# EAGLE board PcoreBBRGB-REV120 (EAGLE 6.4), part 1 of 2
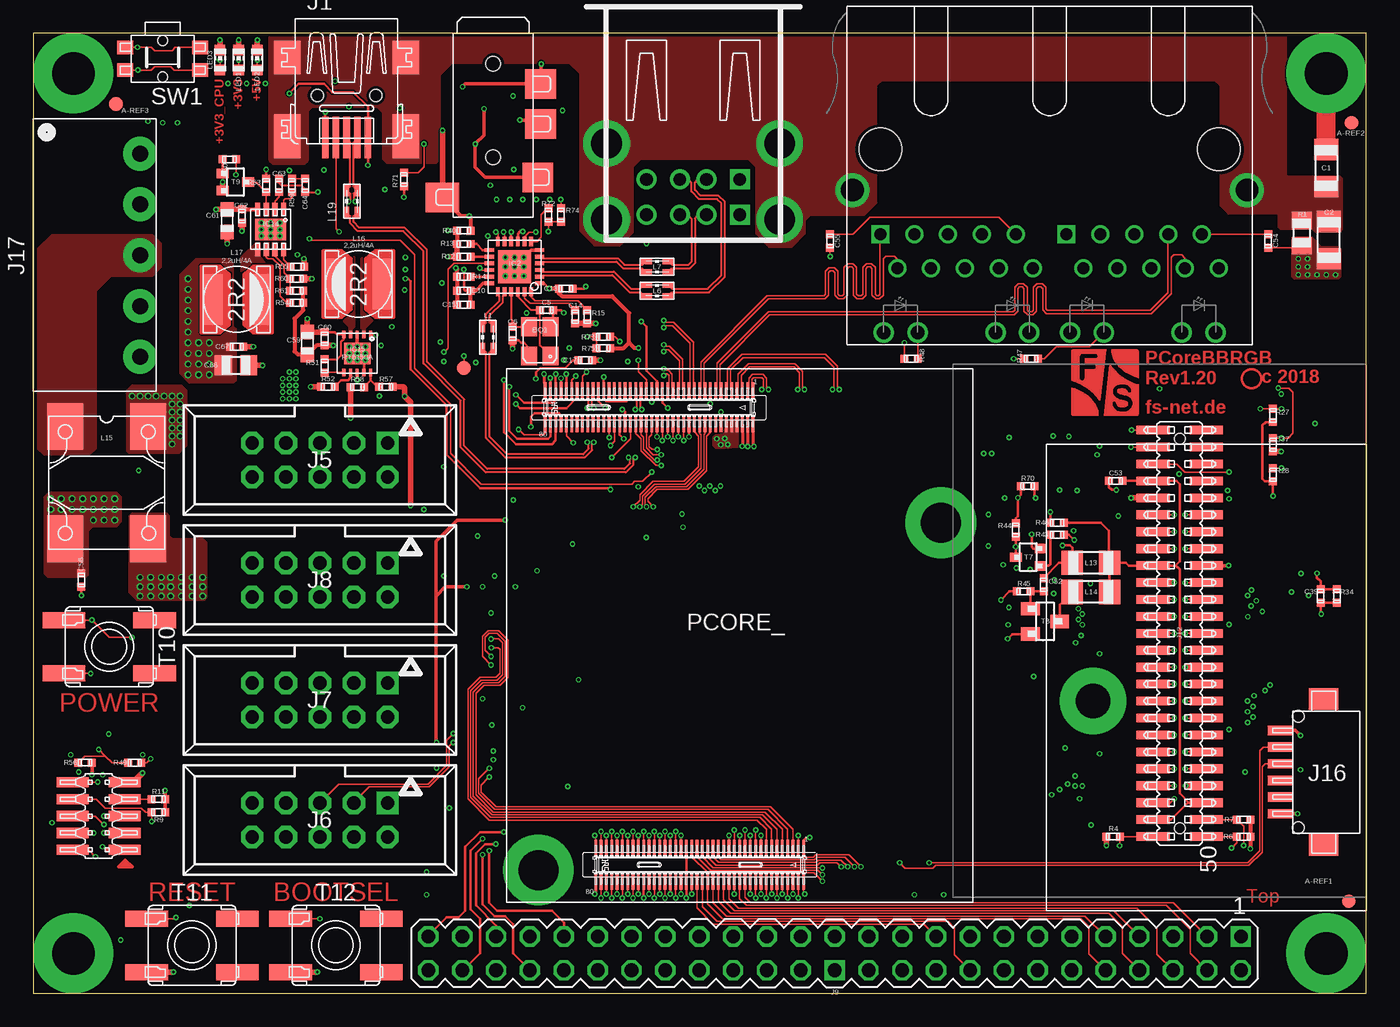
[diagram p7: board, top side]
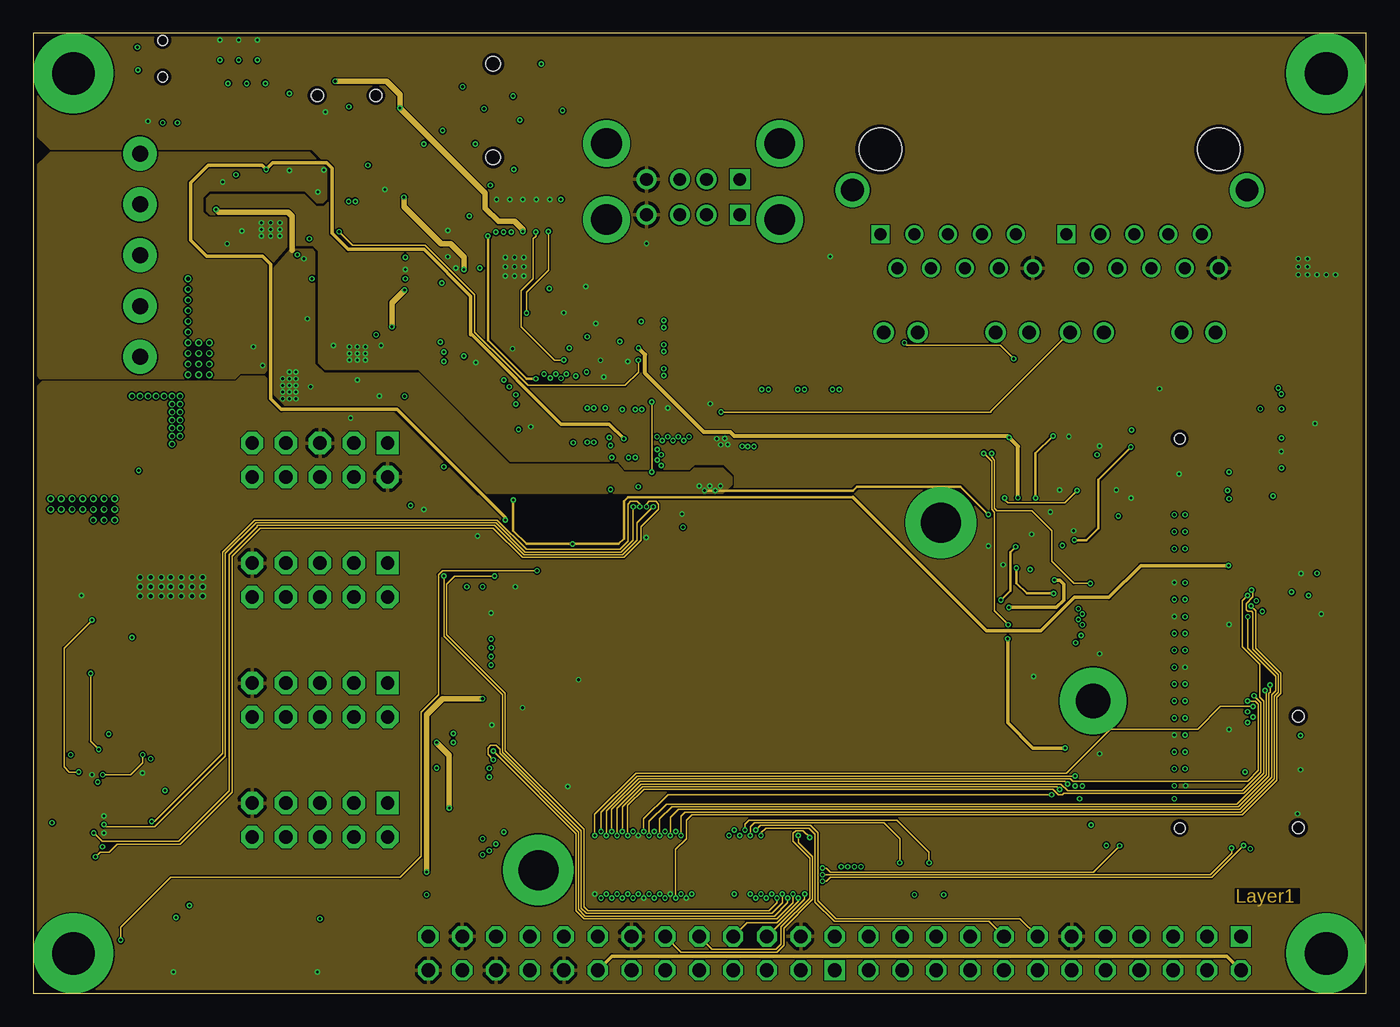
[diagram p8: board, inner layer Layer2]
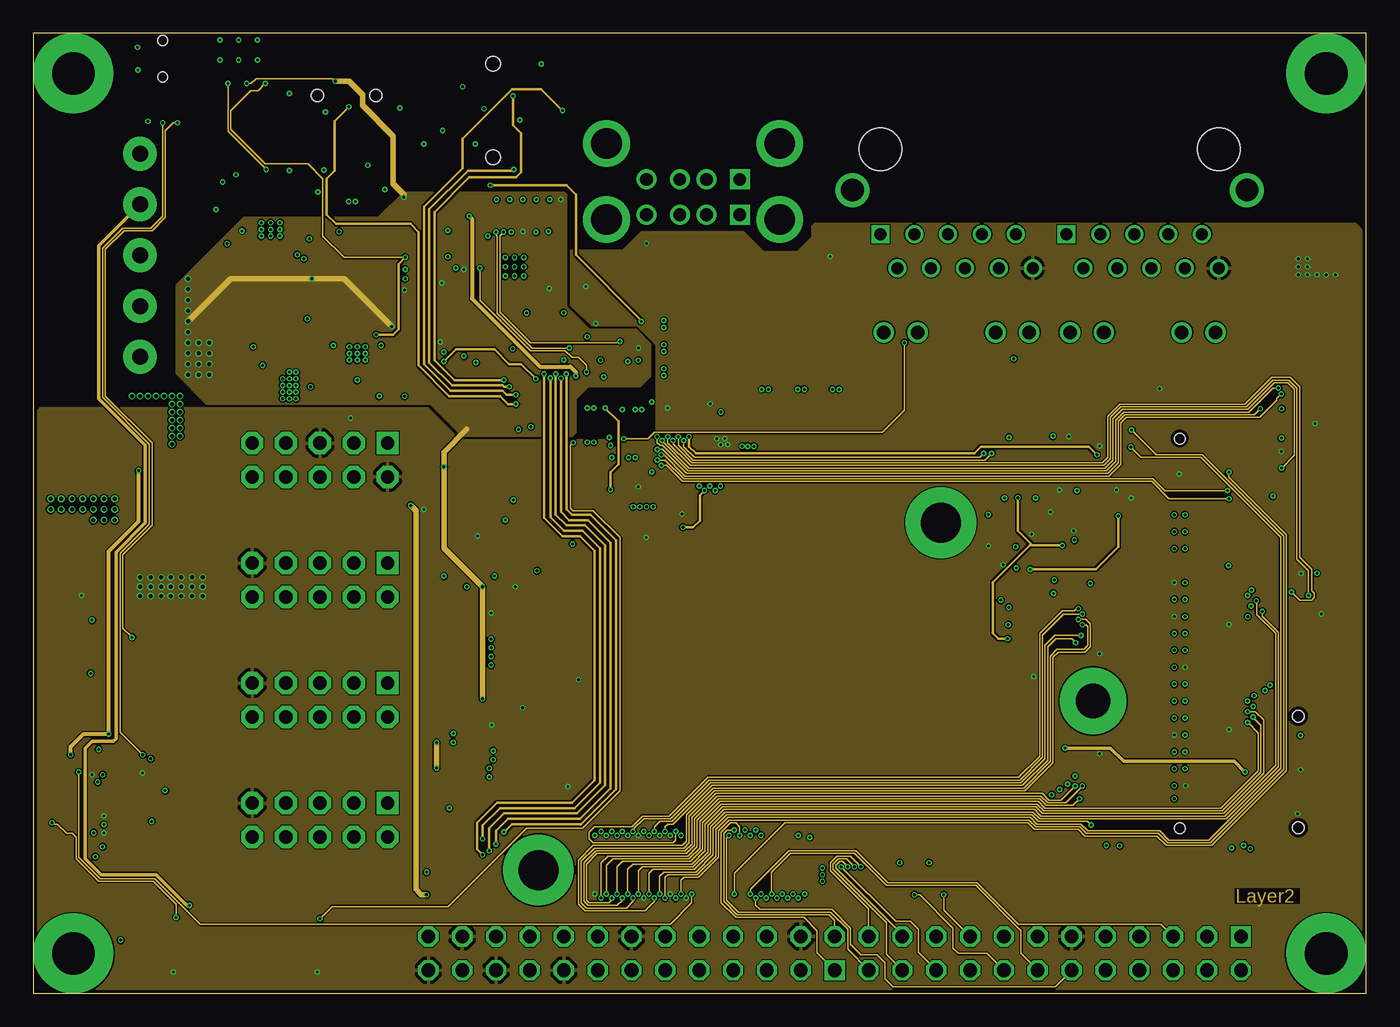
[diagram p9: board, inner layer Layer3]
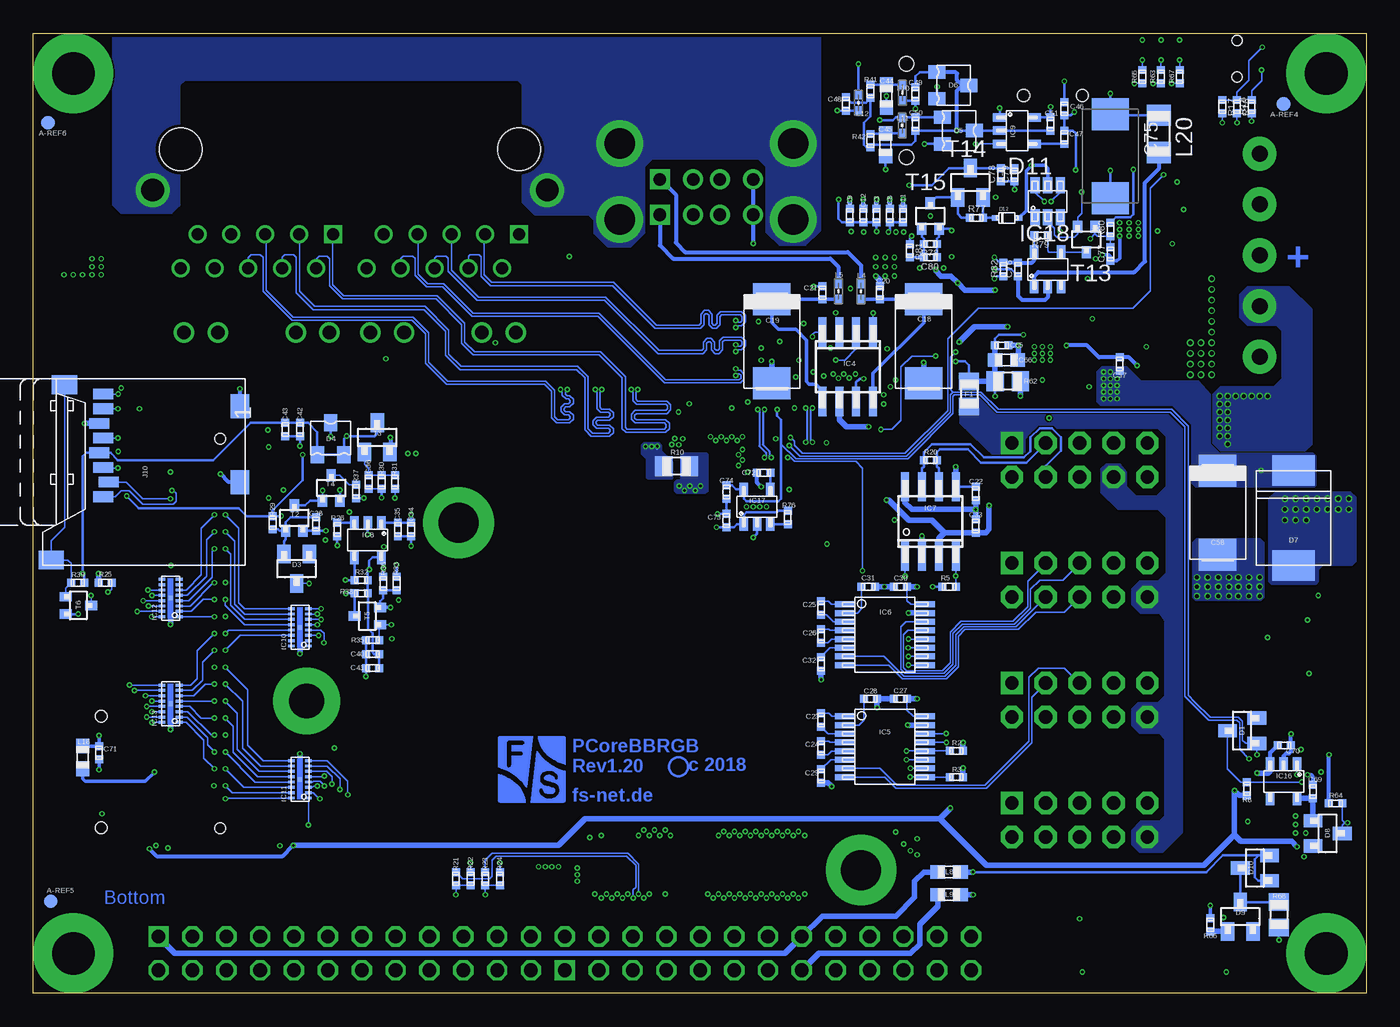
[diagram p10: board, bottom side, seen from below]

Size 100 x 72 mm. Coordinates in mm from the lower left corner, seen from the top.
Outline: 0,0 100,0 100,72 0,72 0,0
Copper layers (1*2*15*16): Top 0.035mm / dielectric 0.14mm / Layer2 0.035mm / dielectric 1.2mm / Layer3 0.035mm / dielectric 0.14mm / Bottom 0.035mm
Design rules "default *": minimum track width 0.1mm, minimum drill 0.2mm, track to track 0.1mm, track to pad 0.1mm, pad to pad 0.1mm, via to via 0.1mm, smd to smd 0.1mm, copper to edge 10mil, drill to drill 8mil, minimum pad ring 0.1mm, minimum via ring 0.1mm, stop-mask expansion 0mil, vias tented up to drill 0.6mm, thermal gap 10mil
Net classes: 0 default: width 0.1 mm, drill 0.2 mm, clearance 0.1 mm; 1 USB: width 0.161 mm, drill 0.2 mm, clearance 0.5 mm to class 0, clearance 0.1 mm; 2 ETHERNET: width 0.127 mm, drill 0.2 mm, clearance 0.5 mm to class 0, clearance 0.5 mm to class 1, clearance 0.1 mm; 3 +3V3: width 0.1 mm, drill 0.2 mm, clearance 0.1 mm to class 0, clearance 0.5 mm to class 1, clearance 0.5 mm to class 2, clearance 0.1 mm

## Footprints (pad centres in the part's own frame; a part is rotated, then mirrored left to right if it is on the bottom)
A-REF = smd 1 x 1: P$1 0,0
FA-238 = smd 1.4 x 1.2: 1 -1.1,-0.8; 2 1.1,-0.8; 3 1.1,0.8; 4 -1.1,0.8
1206 = smd 1.6 x 1.803: 1 -1.4,0; 2 1.4,0
0402@2 = smd 0.6 x 0.6: 1 -0.5,0; 2 0.5,0
SMC_D@1 = smd 2.4 x 2.8: + -3.15,0; - 3.15,0
0603 = smd 1.1 x 1: 1 -0.85,0; 2 0.85,0
0805 = smd 1.3 x 1.5: 1 -0.95,0; 2 0.95,0
SMC_D = smd 2.4 x 2.8: + -3.15,0; - 3.15,0
SOT23 = smd 1 x 1.4: 1 -0.95,-1.1; 2 0.95,-1.1; 3 0,1.1
SOT-23 = smd 1 x 1.27: 1 -1,-1.2; 2 1,-1.2; 3 0,1.2
D-DO214AB(SMC) = smd 2.286 x 3.175: 1 -3.556,0; 2 3.556,0
SOT26 = smd 0.7 x 1.2: 1 -0.95,-1.2; 2 0,-1.2; 3 0.95,-1.2; 4 0.95,1.2; 5 0,1.2; 6 -0.95,1.2
SOD-523 = smd 0.48 x 0.4: 1 -0.9,0; 2 0.9,0
HOLE-3.2X6 = drill 3.2 pad 6: P$1 0,0
SQFN-24 = smd 0.28 x 0.69: 1 -1.25,-1.883; 2 -0.75,-1.883; 3 -0.25,-1.883; 4 0.25,-1.883; 5 0.75,-1.883; 6 1.25,-1.883; 13 1.25,1.883; 14 0.75,1.883; 15 0.25,1.883; 16 -0.25,1.883; 17 -0.75,1.883; 18 -1.25,1.883 | smd 0.69 x 0.28: 7 1.883,-1.25; 8 1.883,-0.75; 9 1.883,-0.25; 10 1.883,0.25; 11 1.883,0.75; 12 1.883,1.25; 19 -1.883,1.25; 20 -1.883,0.75; 21 -1.883,0.25; 22 -1.883,-0.25; 23 -1.883,-0.75; 24 -1.883,-1.25 | smd 2.5 x 2.5: 25 0,0
SO-8$1 = smd 0.6 x 2.2: 1 -1.905,-2.6; 2 -0.635,-2.6; 3 0.635,-2.6; 4 1.905,-2.6; 5 1.905,2.6; 6 0.635,2.6; 7 -0.635,2.6; 8 -1.905,2.6
TSSOP-16 = smd 0.45 x 1.5: 1 -2.275,-3; 2 -1.625,-3; 3 -0.975,-3; 4 -0.325,-3; 5 0.325,-3; 6 0.975,-3; 7 1.625,-3; 8 2.275,-3; 9 2.275,3; 10 1.625,3; 11 0.975,3; 12 0.325,3; 13 -0.325,3; 14 -0.975,3; 15 -1.625,3; 16 -2.275,3
SO-8 = smd 0.6 x 2.2: 1 -1.9,-2.6; 2 -0.635,-2.6; 3 0.635,-2.6; 4 1.9,-2.6; 5 1.9,2.6; 6 0.635,2.6; 7 -0.635,2.6; 8 -1.9,2.6
SOT23-5 = smd 0.635 x 1: 1 -1,-1.3; 2 0,-1.3; 3 1,-1.3; 4 1,1.3; 5 -1,1.3
SOT1168-1 = smd 0.22 x 0.5: 1 -1.4,-0.64; 2 -1,-0.64; 3 -0.6,-0.64; 4 -0.2,-0.64; 5 0.2,-0.64; 6 0.6,-0.64; 7 1,-0.64; 8 1.4,-0.64; 9 1.4,0.64; 10 1,0.64; 11 0.6,0.64; 12 0.2,0.64; 13 -0.2,0.64; 14 -0.6,0.64; 15 -1,0.64; 16 -1.4,0.64 | smd 0.35 x 0.3: 17 0,0
WDFN-8L = smd 0.4 x 1: 1 -0.975,-1.5; 2 -0.325,-1.5; 3 0.325,-1.5; 4 0.975,-1.5; 5 0.975,1.5; 6 0.325,1.5; 7 -0.325,1.5; 8 -0.975,1.5 | smd 2.35 x 1.6: 9 0,0
WDFN-10L3X3 = smd 0.23 x 0.55: 1 -1,-1.425; 2 -0.5,-1.425; 3 0,-1.425; 4 0.5,-1.425; 5 1,-1.425; 6 1,1.425; 7 0.5,1.425; 8 0,1.425; 9 -0.5,1.425; 10 -1,1.425 | smd 2 x 1.6: 11 0,0
SOT23-5@1 = smd 0.635 x 1: 1 -1,-1.3; 2 0,-1.3; 3 1,-1.3; 4 1,1.3; 5 -1,1.3
32005-201 = smd 0.5 x 3.1: 1 1.6,-8.918; 2 0.8,-8.918; 3 0,-8.918; 4 -0.8,-8.918; 5 -1.6,-8.918 | smd 2 x 2.5: M1 -4.45,-2.918; M2 4.45,-2.918 | smd 2 x 3.3: M3 4.45,-8.818; M4 -4.45,-8.818 | hole 0.9: -2.2,-5.768; 2.2,-5.768
10-POL.SMD-127 = smd 0.76 x 2.4: 1 -2.54,-1.95; 2 -2.54,1.95; 3 -1.27,-1.95; 4 -1.27,1.95; 5 0,-1.95; 6 0,1.95; 7 1.27,-1.95; 8 1.27,1.95; 9 2.54,-1.95; 10 2.54,1.95
LUMBERG-2410-03 = drill 0.95 pad 1.5 square: 1 12.96,3.5; 5 15.61,3.5 | drill 0.95 pad 1.5: 2 12.96,1; 3 12.96,-1; 4 12.96,-3.5; 6 15.61,1; 7 15.61,-1; 8 15.61,-3.5 | drill 2.3 pad 3.5: 9 10.26,6.5; 10 10.26,-6.5; 11 15.96,6.5; 12 15.96,-6.5
CON-10POL.-STIFTWANNE = drill 1 pad 1.676 square: 1 -5.08,-1.27 | drill 1 pad 1.676 octagon: 2 -5.08,1.27; 3 -2.54,-1.27; 4 -2.54,1.27; 5 0,-1.27; 6 0,1.27; 7 2.54,-1.27; 8 2.54,1.27; 9 5.08,-1.27; 10 5.08,1.27
50-POL. = drill 1.016 square: 1 -30.48,-1.27; 26 0,1.27 | drill 1.016 octagon: 2 -30.48,1.27; 3 -27.94,-1.27; 4 -27.94,1.27; 5 -25.4,-1.27; 6 -25.4,1.27; 7 -22.86,-1.27; 8 -22.86,1.27; 9 -20.32,-1.27; 10 -20.32,1.27; 11 -17.78,-1.27; 12 -17.78,1.27; 13 -15.24,-1.27; 14 -15.24,1.27; 15 -12.7,-1.27; 16 -12.7,1.27; 17 -10.16,-1.27; 18 -10.16,1.27; 19 -7.62,-1.27; 20 -7.62,1.27; 21 -5.08,-1.27; 22 -5.08,1.27; 23 -2.54,-1.27; 24 -2.54,1.27; 25 0,-1.27; 27 2.54,-1.27; 28 2.54,1.27; 29 5.08,-1.27; 30 5.08,1.27; 31 7.62,-1.27; 32 7.62,1.27; 33 10.16,-1.27; 34 10.16,1.27; 35 12.7,-1.27; 36 12.7,1.27; 37 15.24,-1.27; 38 15.24,1.27; 39 17.78,-1.27; 40 17.78,1.27; 41 20.32,-1.27; 42 20.32,1.27; 43 22.86,-1.27; 44 22.86,1.27; 45 25.4,-1.27; 46 25.4,1.27; 47 27.94,-1.27; 48 27.94,1.27; 49 30.48,-1.27; 50 30.48,1.27
MICRO-SD-PUSHPULL = smd 0.8 x 1.5: 1 -1.85,3.05; 2 -0.75,2.65; 3 0.35,3.05; 4 1.45,3.35; 5 2.55,3.05; 6 3.65,3.35; 7 4.75,3.05; 8 5.85,3.05 | smd 1.4 x 1.9: 9@1 -6.6,6.95; 9@2 6.55,5.95 | smd 1.8 x 1.4: 10@1 -0.75,-7.2; 10@2 4.95,-7.2
CON-AUDIO-SJ2 = smd 2.2 x 2.5: 1 6,-3.81 | smd 2.2 x 2.3: 2 4.5,3.35; 3 0.5,3.55; 4 -2.5,3.55 | hole 1.1: -4,0; 3,0
CON-DISPLAY-50-PCORE = smd 0.65 x 2.5: 1 15.24,2; 2 15.24,-2; 3 13.97,2; 4 13.97,-2; 5 12.7,2; 6 12.7,-2; 7 11.43,2; 8 11.43,-2; 9 10.16,2; 10 10.16,-2; 11 8.89,2; 12 8.89,-2; 13 7.62,2; 14 7.62,-2; 15 6.35,2; 16 6.35,-2; 17 5.08,2; 18 5.08,-2; 19 3.81,2; 20 3.81,-2; 21 2.54,2; 22 2.54,-2; 23 1.27,2; 24 1.27,-2; 25 0,2; 26 0,-2; 27 -1.27,2; 28 -1.27,-2; 29 -2.54,2; 30 -2.54,-2; 31 -3.81,2; 32 -3.81,-2; 33 -5.08,2; 34 -5.08,-2; 35 -6.35,2; 36 -6.35,-2; 37 -7.62,2; 38 -7.62,-2; 39 -8.89,2; 40 -8.89,-2; 41 -10.16,2; 42 -10.16,-2; 43 -11.43,2; 44 -11.43,-2; 45 -12.7,2; 46 -12.7,-2; 47 -13.97,2; 48 -13.97,-2; 49 -15.24,2; 50 -15.24,-2 | drill 2.6 pad 5: P$1 -5.08,6.5 | hole 0.8: 14.605,0; -14.605,0
TRJG27440ADNL = drill 0.9 square: L1 -1.27,-2.54; R1 12.7,-2.54 | drill 0.9: L2 -2.54,0; L3 -3.81,-2.54; L4 -5.08,0; L5 -6.35,-2.54; L6 -7.62,0; L7 -8.89,-2.54; L8 -10.16,0; L9 -11.43,-2.54; L10 -12.7,0; R2 11.43,0; R3 10.16,-2.54; R4 8.89,0; R5 7.62,-2.54; R6 6.35,0; R7 5.08,-2.54; R8 3.81,0; R9 2.54,-2.54; R10 1.27,0 | drill 1.02: L11 -1.525,4.83; L12 -4.065,4.83; L13 -9.905,4.83; L14 -12.445,4.83; R11 12.445,4.83; R12 9.905,4.83; R13 4.065,4.83; R14 1.525,4.83 | drill 1.7: SHIELD1 -14.8,-5.84; SHIELD2 14.8,-5.84 | hole 3.2: -12.7,-8.89; 12.7,-8.89
CON-HIROSE-DF13A-6P = smd 0.7 x 1.8: 1 -3.125,-6; 2 -1.875,-6; 3 -0.625,-6; 4 0.625,-6; 5 1.875,-6; 6 3.125,-6 | smd 1.6 x 2.2: 7 -5.475,-2.7; 8 5.475,-2.7 | hole 0.9: -4.175,-4.6; 4.175,-4.6
CON-5-POL. = drill 1.2 pad 2.54: 1 7.62,-8; 2 3.81,-8; 3 0,-8; 4 -3.81,-8; 5 -7.62,-8
WE-CNSW_0805 = smd 0.4 x 0.9: 1 -0.4,-0.85; 2 -0.4,0.85; 3 0.4,0.85; 4 0.4,-0.85
0402 = smd 0.7 x 0.6: 1 -0.6,0; 2 0.6,0
L-WE-SL5 = smd 3.5 x 2.7: 1 4.21,3.11; 2 -4.21,3.11; 3 -4.21,-3.11; 4 4.21,-3.11
VLC5045 = smd 1.4 x 3.8: 1 -1.79,0; 2 1.76,0
LED0603 = smd 0.8 x 0.8: A 0,-0.75; C 0,0.75
PICOCORE = smd 0.2 x 1.14: J1-1 4.8,-15.895; J1-2 4.8,-18.505; J1-3 4.4,-15.895; J1-4 4.4,-18.505; J1-5 4,-15.895; J1-6 4,-18.505; J1-7 3.6,-15.895; J1-8 3.6,-18.505; J1-9 3.2,-15.895; J1-10 3.2,-18.505; J1-11 2.8,-15.895; J1-12 2.8,-18.505; J1-13 2.4,-15.895; J1-14 2.4,-18.505; J1-15 2,-15.895; J1-16 2,-18.505; J1-17 1.6,-15.895; J1-18 1.6,-18.505; J1-19 1.2,-15.895; J1-20 1.2,-18.505; J1-21 0.8,-15.895; J1-22 0.8,-18.505; J1-23 0.4,-15.895; J1-24 0.4,-18.505; J1-25 0,-15.895; J1-26 0,-18.505; J1-27 -0.4,-15.895; J1-28 -0.4,-18.505; J1-29 -0.8,-15.895; J1-30 -0.8,-18.505; J1-31 -1.2,-15.895; J1-32 -1.2,-18.505; J1-33 -1.6,-15.895; J1-34 -1.6,-18.505; J1-35 -2,-15.895; J1-36 -2,-18.505; J1-37 -2.4,-15.895; J1-38 -2.4,-18.505; J1-39 -2.8,-15.895; J1-40 -2.8,-18.505; J1-41 -3.2,-15.895; J1-42 -3.2,-18.505; J1-43 -3.6,-15.895; J1-44 -3.6,-18.505; J1-45 -4,-15.895; J1-46 -4,-18.505; J1-47 -4.4,-15.895; J1-48 -4.4,-18.505; J1-49 -4.8,-15.895; J1-50 -4.8,-18.505; J1-51 -5.2,-15.895; J1-52 -5.2,-18.505; J1-53 -5.6,-15.895; J1-54 -5.6,-18.505; J1-55 -6,-15.895; J1-56 -6,-18.505; J1-57 -6.4,-15.895; J1-58 -6.4,-18.505; J1-59 -6.8,-15.895; J1-60 -6.8,-18.505; J1-61 -7.2,-15.895; J1-62 -7.2,-18.505; J1-63 -7.6,-15.895; J1-64 -7.6,-18.505; J1-65 -8,-15.895; J1-66 -8,-18.505; J1-67 -8.4,-15.895; J1-68 -8.4,-18.505; J1-69 -8.8,-15.895; J1-70 -8.8,-18.505; J1-71 -9.2,-15.895; J1-72 -9.2,-18.505; J1-73 -9.6,-15.895; J1-74 -9.6,-18.505; J1-75 -10,-15.895; J1-76 -10,-18.505; J1-77 -10.4,-15.895; J1-78 -10.4,-18.505; J1-79 -10.8,-15.895; J1-80 -10.8,-18.505; J2-1 1,18.405; J2-2 1,15.795; J2-3 0.6,18.405; J2-4 0.6,15.795; J2-5 0.2,18.405; J2-6 0.2,15.795; J2-7 -0.2,18.405; J2-8 -0.2,15.795; J2-9 -0.6,18.405; J2-10 -0.6,15.795; J2-11 -1,18.405; J2-12 -1,15.795; J2-13 -1.4,18.405; J2-14 -1.4,15.795; J2-15 -1.8,18.405; J2-16 -1.8,15.795; J2-17 -2.2,18.405; J2-18 -2.2,15.795; J2-19 -2.6,18.405; J2-20 -2.6,15.795; J2-21 -3,18.405; J2-22 -3,15.795; J2-23 -3.4,18.405; J2-24 -3.4,15.795; J2-25 -3.8,18.405; J2-26 -3.8,15.795; J2-27 -4.2,18.405; J2-28 -4.2,15.795; J2-29 -4.6,18.405; J2-30 -4.6,15.795; J2-31 -5,18.405; J2-32 -5,15.795; J2-33 -5.4,18.405; J2-34 -5.4,15.795; J2-35 -5.8,18.405; J2-36 -5.8,15.795; J2-37 -6.2,18.405; J2-38 -6.2,15.795; J2-39 -6.6,18.405; J2-40 -6.6,15.795; J2-41 -7,18.405; J2-42 -7,15.795; J2-43 -7.4,18.405; J2-44 -7.4,15.795; J2-45 -7.8,18.405; J2-46 -7.8,15.795; J2-47 -8.2,18.405; J2-48 -8.2,15.795; J2-49 -8.6,18.405; J2-50 -8.6,15.795; J2-51 -9,18.405; J2-52 -9,15.795; J2-53 -9.4,18.405; J2-54 -9.4,15.795; J2-55 -9.8,18.405; J2-56 -9.8,15.795; J2-57 -10.2,18.405; J2-58 -10.2,15.795; J2-59 -10.6,18.405; J2-60 -10.6,15.795; J2-61 -11,18.405; J2-62 -11,15.795; J2-63 -11.4,18.405; J2-64 -11.4,15.795; J2-65 -11.8,18.405; J2-66 -11.8,15.795; J2-67 -12.2,18.405; J2-68 -12.2,15.795; J2-69 -12.6,18.405; J2-70 -12.6,15.795; J2-71 -13,18.405; J2-72 -13,15.795; J2-73 -13.4,18.405; J2-74 -13.4,15.795; J2-75 -13.8,18.405; J2-76 -13.8,15.795; J2-77 -14.2,18.405; J2-78 -14.2,15.795; J2-79 -14.6,18.405; J2-80 -14.6,15.795 | drill 3 pad 5.3: P$1 -15.1,-17.6; P$2 15.1,8.45
0402' = smd 0.6 x 0.6: 1 -0.5,0; 2 0.5,0
TASTER-WE-436351045816 = smd 1.2 x 1: 1 2.8,0.85; 2 2.8,-0.85; 3 -2.8,0.85; 4 -2.8,-0.85 | hole 0.75: 0,-1.375; 0,1.375
SOT323(SC70) = smd 0.7 x 0.9: 1 -0.65,-0.95; 2 0.65,-0.95; 3 0,0.95
TASTER_SMD = smd 3.2 x 1.2: 11 -3.4,-2; 12 3.4,-2; 21 -3.4,2; 22 3.4,2
TEST2 = smd 1 x 1: P$1 0,0

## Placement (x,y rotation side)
A-REF1  [A-REF]  98.7,6.9 0 top
A-REF2  [A-REF]  98.9,65.3 0 top
A-REF3  [A-REF]  6.2,66.7 0 top
A-REF4  [A-REF]  6.2,66.7 0 bottom
A-REF5  [A-REF]  98.7,6.9 0 bottom
A-REF6  [A-REF]  98.9,65.3 0 bottom
BQ1  24MHz  [FA-238]  38,48.9 90 top
C1  1nF/2kV  [1206]  97,61.9 90 top
C2  1nF/2kV  [1206]  97.2,56.5 270 top
C3  0.1uF  [0402@2]  36.73,58.34 90 bottom
C5  22pF  [0402@2]  38.5,51.25 180 top
C6  22pF  [0402@2]  35.95,49.5 90 top
C8  1nF  [0402@2]  35.74,58.34 90 bottom
C9  1nF  [0402@2]  38.74,58.34 90 bottom
C10  0.1uF  [0402@2]  32.3,52.7 180 top
C11  1uF  [0402@2]  34.75,58.34 90 bottom
C12  1uF  [0402@2]  37.73,58.34 90 bottom
C13  0.1uF  [0402@2]  39.94,52.86 0 top
C14  0.1uF  [0402@2]  40.65,50.75 270 top
C15  1nF  [0402@2]  32.3,51.65 180 top
C17  0.1µF  [0402@2]  41.4,47.48 180 top
C18  220µF  [SMC_D@1]  33.2,48.9 270 bottom
C19  220µF  [SMC_D@1]  44.6,48.9 270 bottom
C20  0.1uF  [0402@2]  36.5,52.55 270 bottom
C21  0.1uF  [0402@2]  40.8,52.55 270 bottom
C22  0.1uF  [0402@2]  29.3,37.5 270 bottom
C23  0.1uF  [0402@2]  40.9,20.5 270 bottom
C24  0.1uF  [0402@2]  40.9,18.4 270 bottom
C25  0.1uF  [0402@2]  40.9,28.9 270 bottom
C26  0.1uF  [0402@2]  40.9,26.8 270 bottom
C27  0.1uF  [0402@2]  34.95,22.1 180 bottom
C28  0.1uF  [0402@2]  37.2,22.1 0 bottom
C29  0.1uF  [0402@2]  40.9,16.3 270 bottom
C30  0.1uF  [0402@2]  34.94,30.5 180 bottom
C31  0.1uF  [0402@2]  37.36,30.5 0 bottom
C32  0.1uF  [0402@2]  40.9,24.7 270 bottom
C33  0.1uF  [0402@2]  29.3,35.05 90 bottom
C34  10uF  [0402@2]  71.65,34.8 270 bottom
C35  0.1uF  [0402@2]  72.65,34.8 270 bottom
C36  0.1uF  [0402@2]  74.85,38.34 90 bottom
C37  22pF  [0402@2]  93,41.15 270 top
C38  0.1uF  [0402@2]  78.8,35.2 270 bottom
C39  0.1uF  [0402@2]  96.58,29.8 270 top
C40  10uF  [0402@2]  74.55,25.45 180 bottom
C41  10uF  [0402@2]  74.55,24.4 180 bottom
C42  10uF  [0402@2]  80,42.29 270 bottom
C43  0.1uF  [0402@2]  81.1,42.29 270 bottom
C44  22uF  [0603]  35.99,67.3 90 bottom
C45  22uF  [0603]  36.06,63.65 90 bottom
C46  10uF  [0402@2]  22.64,66.35 270 bottom
C47  10uF  [0402@2]  22.64,64.2 90 bottom
C48  12pF  [0402@2]  39.03,66.7 90 bottom
C49  220pF  [0402@2]  33.82,67.45 270 bottom
C50  220pF  [0402@2]  33.81,65.2 270 bottom
C51  10uF  [0402@2]  23.68,65.2 270 bottom
C52  0.1uF  [0402@2]  75.8,30.64 270 top
C53  0.1uF  [0402@2]  81.21,38.43 180 top
C54  0.1uF  [0402@2]  92.64,56.43 270 top
C55  0.1uF  [0402@2]  59.78,56.43 270 top
C56  0.1uF  [0402@2]  3.6,31 270 top
C57  0.1uF  [0402@2]  18.5,47.2 90 bottom
C58  220µF  [SMC_D@1]  11.15,36.05 270 bottom
C59  10uF  [0603]  20.55,48.75 270 top
C60  0.1uF  [0402@2]  21.85,49.1 270 top
C61  10uF  [0603]  14.54,57.95 270 top
C62  0.1uF  [0402@2]  15.66,58.3 270 top
C63  100pF  [0402@2]  18.43,60.6 90 top
C64  560pF  [0402@2]  20.4,60.6 270 top
C65  0.1uF  [0402@2]  27.35,48.6 0 bottom
C66  10uF  [0603]  27,47.5 0 bottom
C67  0.1uF  [0402@2]  15.25,48.5 0 top
C68  22uF  [0805]  15.2,47.1 0 top
C69  0.1uF  [0402@2]  4,15.15 90 bottom
C70  0.1uF  [0402@2]  6.15,18.6 180 bottom
C71  0.1uF  [0402@2]  95.07,18.05 270 bottom
C72  10uF  [0402@2]  45.2,39.04 180 bottom
C73  10uF  [0402@2]  48.01,35.46 90 bottom
C74  10uF  [0402@2]  48,37.6 270 bottom
C75  220µF  [SMC_D]  19.2,62.8 270 bottom
C76  0.1uF  [0402@2]  26.12,54.3 90 bottom
C77  0.1uF  [0402@2]  19.18,55.45 90 bottom
C78  0.1uF  [0402@2]  27.4,61.4 90 bottom
C79  10uF  [0402@2]  26.38,61.4 90 bottom
C80  0.1uF  [0402@2]  32.7,55.19 180 bottom
D1  BAT54C  [SOT23]  9.31,19.7 90 bottom
D3  BAT54C  [SOT23]  80.25,31.85 180 bottom
D4  PGB102ST23  [SOT-23]  77.69,41.59 0 bottom
D5  PGB102ST23  [SOT-23]  30.6,64.7 270 bottom
D6  PGB102ST23  [SOT-23]  31,68.1 270 bottom
D7  SK56L  [D-DO214AB(SMC)]  5.45,35.65 270 bottom
D8  BAT54C  [SOT23]  2.9,12 270 bottom
D9  BAT54C  [SOT23]  9.45,5.75 0 bottom
D10  BAT54C  [SOT23]  8.35,9.4 90 bottom
D11  B.EMVSUP.2  [SOT26]  23.9,59.4 0 bottom
D12  RB521S30T1G  [SOD-523]  26.94,58.16 0 bottom
F1  1.1A  [0805]  29.79,44.95 270 bottom
H1  HOLE-3.2X6  [HOLE-3.2X6]  3,69 0 top
H2  HOLE-3.2X6  [HOLE-3.2X6]  3,3 0 top
H3  HOLE-3.2X6  [HOLE-3.2X6]  97,3 0 top
H4  HOLE-3.2X6  [HOLE-3.2X6]  97,69 0 top
IC2  USB2422  [SQFN-24]  36.1,54.5 90 top
IC4  MIC2026-1  [SO-8$1]  38.9,47 180 bottom
IC5  SP3232EEY  [TSSOP-16]  36.1,18.5 270 bottom
IC6  SP3232EEY  [TSSOP-16]  36.1,26.9 270 bottom
IC7  TJA1051T/3  [SO-8]  32.7,35.4 0 bottom
IC8  ADP171  [SOT23-5]  74.9,34 180 bottom
IC9  LDO 3V  [SOT23-5]  26.2,64.7 270 bottom
IC10  IP4254CZ16  [SOT1168-1]  80,27.45 90 bottom
IC11  IP4254CZ16  [SOT1168-1]  80,16.05 90 bottom
IC12  IP4254CZ16  [SOT1168-1]  89.7,29.65 90 bottom
IC13  IP4254CZ16  [SOT1168-1]  89.7,21.72 90 bottom
IC14  RT8070  [WDFN-8L]  17.8,57.3 180 top
IC15  RT6150A  [WDFN-10L3X3]  24.3,48 180 top
IC16  NCP303  [SOT23-5]  6.2,15.9 180 bottom
IC17  LDO 3.3V  [SOT23-5]  45.7,36.5 0 bottom
IC18  TPS2051BDBV  [SOT23-5@1]  23.9,54.3 0 bottom
J1  [32005-201]  23.5,73.1 0 top
J2  [10-POL.SMD-127]  4.9,13.3 90 top
J4  [LUMBERG-2410-03]  49.5,74 270 top
J5  [CON-10POL.-STIFTWANNE]  21.5,40 180 top
J6  [CON-10POL.-STIFTWANNE]  21.5,13 180 top
J7  [CON-10POL.-STIFTWANNE]  21.5,22 180 top
J8  [CON-10POL.-STIFTWANNE]  21.5,31 180 top
J9  CON-50-POL.  [50-POL.]  60.12,3 180 top
J10  [MICRO-SD-PUSHPULL]  91.7,39.1 90 bottom
J11  CON-AUDIO-HP-MIC  [CON-AUDIO-SJ2]  34.5,65.7 270 top
J12  [CON-DISPLAY-50-PCORE]  86,27 90 top
J15  [TRJG27440ADNL]  76.25,54.4 180 top
J16  [CON-HIROSE-DF13A-6P]  99.5,16.6 270 top
J17  CON-5-POL.-381  [CON-5-POL.]  0,55.36 90 top
L1  2x90Ohm  [WE-CNSW_0805]  34.1,49.2 0 top
L4  120R/100MHz  [0402]  37.9,52.65 90 bottom
L5  120R/100MHz  [0402]  39.6,52.65 90 bottom
L6  2x90Ohm  [WE-CNSW_0805]  46.8,52.7 270 top
L7  2x90Ohm  [WE-CNSW_0805]  46.8,54.5 270 top
L8  120R/100MHz  [0603]  31.3,9.1 180 bottom
L9  120R/100MHz  [0603]  31.3,7.4 0 bottom
L10  120R@100MHz  [0402]  34.8,67.55 270 bottom
L11  120R@100MHz  [0402]  34.81,65.1 90 bottom
L12  120R@100MHz  [0402]  38.1,66.8 90 bottom
L13  700R/90MHz  [1206]  79.34,32.28 0 top
L14  700R/90MHz  [1206]  79.34,30.1 0 top
L15  [L-WE-SL5]  5.5,38.3 90 top
L16  2,2uH/4A  [VLC5045]  24.4,53.2 0 top
L17  2,2uH/4A  [VLC5045]  15.25,52.05 180 top
L18  120R/100MHz  [0603]  96.3,17.7 270 bottom
L19  2x90Ohm  [WE-CNSW_0805]  23.9,59.4 0 top
L20  700R/90MHz  [1206]  15.56,64.46 270 bottom
LED1  [LED0603]  15.4,70 0 top
LED2  [LED0603]  16.8,70 0 top
LED3  [LED0603]  14,70 0 top
PCORE_  PICOCORE  [PICOCORE]  52.99,26.84 0 top
R1  0R  [0805]  95.15,57.02 270 top
R2  100k  [0402']  30.75,18.18 180 bottom
R3  100k  [0402']  30.75,16.22 180 bottom
R4  100k  [0402']  81,11.76 0 top
R5  100k  [0402']  31.3,30.5 0 bottom
R6  4.7k  [0402']  90.8,11.75 180 top
R7  4.7k  [0402']  90.8,13.03 180 top
R8  10k  [0402@2]  8.95,15.34 270 bottom
R9  10k  [0402@2]  9.38,13.58 0 top
R10  0R01  [0805]  51.75,39.53 180 bottom
R11  10k  [0402@2]  9.38,14.57 0 top
R12  10k  [0402']  32.3,55.25 0 top
R13  10k  [0402']  32.3,56.2 0 top
R14  100k  [0402']  32.3,53.75 0 top
R15  12k  [0402']  41.55,50.75 90 top
R16  0R  [0402']  9.7,66.5 270 bottom
R17  0R  [0402']  10.8,66.5 270 bottom
R18  1k  [0402']  8.6,66.5 90 bottom
R20  120R  [0402']  32.7,40 0 bottom
R21  0R  [0402']  68.3,8.6 90 bottom
R22  0R  [0402']  67.2,8.6 90 bottom
R23  0R  [0402']  66.1,8.6 90 bottom
R24  0R  [0402']  65,8.6 90 bottom
R25  1K  [0402']  94.61,30.8 180 bottom
R26  100K  [0402']  77.2,34.8 90 bottom
R27  10K  [0402@2]  93,43.35 270 top
R28  10K  [0402@2]  93,38.9 270 top
R29  10K  [0402@2]  82.05,35.3 90 bottom
R30  47K  [0402@2]  73.87,38.34 270 bottom
R31  10K  [0402@2]  72.87,38.34 90 bottom
R32  14K  [0402@2]  75.4,31 0 bottom
R33  2K49  [0402@2]  72.75,30.74 270 bottom
R34  100K  [0402@2]  97.81,29.8 90 top
R35  100K  [0402@2]  74.55,26.5 0 bottom
R36  0R  [0402']  73.75,30.74 90 bottom
R37  49R9  [0402@2]  75.8,37.65 270 bottom
R38  11.8K  [0402@2]  75.4,30 0 bottom
R39  10K  [0402@2]  96.67,30.79 0 bottom
R40  0R  [0402@2]  32.3,57.2 0 top
R41  10k  [0402@2]  37.2,67.65 270 bottom
R42  10k  [0402@2]  37.2,63.95 90 bottom
R43  4k7  [0402']  76.8,34.4 180 top
R44  22k  [0402']  73.7,34.76 90 top
R45  47k  [0402']  74.31,30.14 0 top
R46  100k  [0402@2]  76.8,35.3 0 top
R47  300R  [0402']  74.85,47.6 0 top
R48  300R  [0402']  65.85,47.6 180 top
R49  1k  [0402']  7.6,17.3 180 top
R50  1k  [0402']  14.7,62.55 180 top
R51  100k  [0402']  21.85,47.05 270 top
R52  100k  [0402']  22.1,45.5 0 top
R53  100k  [0402']  17.47,60.6 270 top
R54  10k  [0402']  19.75,51.8 180 top
R55  47k  [0402']  19.8,54.5 180 top
R56  1k  [0402']  3.88,17.31 180 top
R57  150k  [0402@2]  26.45,45.48 0 top
R58  16.5k  [0402@2]  24.3,45.47 0 top
R59  30k1  [0402@2]  19.41,60.6 270 top
R60  75k  [0402@2]  19.75,53.6 0 top
R61  24k  [0402@2]  19.75,52.69 180 top
R62  0R  [0805]  26.9,45.9 180 bottom
R63  150R  [0402@2]  15.4,68.75 270 bottom
R64  10k  [0402@2]  2.3,14.25 180 bottom
R65  221R  [0402@2]  16.8,68.75 270 bottom
R66  10k  [0402']  11.7,5.15 90 bottom
R67  150R  [0402@2]  14,68.75 270 bottom
R68  0,01R  [0805]  6.55,5.9 270 bottom
R70  0R  [0402']  74.59,38.05 0 top
R71  0R  [0402']  27.8,61.05 90 top
R72  0R  [0402']  38.64,58.37 270 top
R73  0R  [0402']  42.75,49.24 180 top
R74  10k  [0402@2]  39.58,58.37 90 top
R75  10k  [0402@2]  42.76,48.39 0 top
R76  0R  [0402']  43.39,35.69 270 bottom
R77  10k  [0402@2]  29.25,58.16 0 bottom
R78  100k  [0402@2]  32.7,56.2 180 bottom
R79  10k  [0402@2]  24.4,56.84 180 bottom
R80  10k  [0402@2]  19.18,57.28 90 bottom
R81  10k  [0402']  34.25,55.69 270 bottom
R82  0R  [0402']  27.21,54.3 90 bottom
SW1  [TASTER-WE-436351045816]  9.7,70.1 180 top
T2  BSS138W  [SOT323(SC70)]  80.42,35.65 0 bottom
T3  SI2301DS  [SOT23]  74.2,41.69 0 bottom
T4  BSS138W  [SOT323(SC70)]  77.65,37.9 0 bottom
T5  BSS138W  [SOT323(SC70)]  74.95,28.3 90 bottom
T6  BSS138W  [SOT323(SC70)]  96.62,29.1 270 bottom
T7  BSS138  [SOT323(SC70)]  74.65,32.71 90 top
T8  SI2301  [SOT23]  75.9,27.9 270 top
T9  BSS138W  [SOT323(SC70)]  15.15,60.85 270 top
T10  [TASTER_SMD]  5.7,26 0 top
T11  [TASTER_SMD]  11.9,3.6 0 top
T12  [TASTER_SMD]  22.7,3.6 0 top
T13  BSS138W  [SOT323(SC70)]  21,56.55 180 bottom
T14  SI2301  [SOT23]  29.7,60.8 0 bottom
T15  BSS138W  [SOT323(SC70)]  32.7,58.3 0 bottom
TP1  [TEST2]  32.3,46.9 0 top
U$31  [F&S-LOGO-NEU-200]  80.4,45.8 0 top
U$35  [F&S-LOGO-NEU-200]  62.6,16.8 0 bottom

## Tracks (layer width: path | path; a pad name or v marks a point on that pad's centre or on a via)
!BOOTSEL  (via drill 0.2)
  Top 0.1: PCORE_.J2-72 39.99,41.81 v40.5,41.3 | v21.5,5.6 T12.21
  Layer3 0.1: v21.5,5.6 22.4,6.5 31.1,6.5 37,12.4 41.2,12.4 44,15.2 44,34.2 42,36.2 40.5,36.2 40.3,36.4 40.3,41.1 v40.5,41.3
!ETH_A_LED  (via drill 0.2)
  Top 0.1: PCORE_.J2-14 v51.59,43.6
  Layer2 0.1: v51.59,43.6 71.86,43.6 71.86,43.65 J15.L11
!JTAG_SRST  (via drill 0.2)
  Top 0.1: J2.10 v4.83,15.84
  Bottom 0.1: v4.83,15.84 R8.1 9.42,15.84 10.41,16.83 D1.3
!RESET_BTN  (via drill 0.2)
  Top 0.1: T11.21 10.6,5.6 v10.7,5.7
  Layer3 0.1: v10.7,5.7 10.7,6.7 9,8.4 4.9,8.4 3.2,10.1 3.2,11.7 2.9,12 2.5,12 1.8,12.7 1.5,12.7 v1.4,12.8
  Bottom 0.1: v1.4,12.8 1.6,12.8 | 1.6,12.8 1.8,12.6 D8.3 | 1.6,12.8 1.8,13 R64.1
!RESET_IN  (via drill 0.2, 0.2 pad 0.25)
  Top 0.1: IC2.15 31.55,54.75 31.1,54.3 31.1,48.4 v30.8,48.1 | v43.3,41.1 43.6,41.4 PCORE_.J2-54
  Layer2 0.1: v5.2,16.4 7.3,16.4 8.2,17.3 v8.2,17.9
  Layer3 0.1: v9.7,65.3 9.7,58.3 8.8,57.4 6.7,57.4 5.2,55.9 5.2,44.7 8.7,41.2 8.7,35.2 6.5,33 6.5,19.6 v8.2,17.9
  Bottom 0.1: 31,45.1 31.2,44.9 31.2,43.6 34.5,40.3 42.5,40.3 v43.3,41.1 | 31,45.1 28.9,45.1 27.6,43.8 14.6,43.8 13.35,42.55 13.35,22.36 12.84,21.85 12.84,21.84 11.7,20.7 9.6,20.7 9.3,20.4 9.3,19 9.05,18.75 D1.1 v8.2,17.9 | v30.8,48.1 31.2,47.7 31.2,45.3 31,45.1 | IC16.1 v5.2,16.4 | R16.2 v9.7,65.3
!USB1_OC  (via drill 0.2)
  Top 0.1: IC2.8 36.85,56.75 37.2,57.1 v37.7,57.1
  Layer2 0.1: v37.7,57.1 37.7,56.8 37.5,56.6 37.5,53.6 36.6,52.7 36.6,50 39.1,47.5 v39.8,47.5
  Bottom 0.1: v39.8,47.5 39.1,47.5 38.27,48.34 IC4.2
!USB2_OC  (via drill 0.2)
  Top 0.1: 34.78,57.02 v34.7,57.1 | 34.82,56.98 v34.7,57.1 | IC2.12 34.85,56.95 v34.7,57.1
  Layer3 0.1: v34.7,57.1 34.7,56.9 34.8,56.8 34.8,51 37.4,48.4 v40.2,48.4
  Bottom 0.1: v40.2,48.4 39.9,48.4 39.53,48.77 IC4.3
!USB_OTG_PWR  (via drill 0.2)
  Top 0.1: v46.39,44.36 PCORE_.J2-39 | v20.7,56.6 20.8,56.5 27.5,56.5 28.6,55.4 28.6,46.9 31.3,44.2 31.3,40.5 33.6,38.2 44.9,38.2 45.1,38.4 45.7,38.4 v46.4,39.1
  Layer2 0.1: v46.4,39.1 v46.4,44.35 v46.39,44.36
  Bottom 0.1: C77.2 R80.1 20.18,56.78 20.35,56.95 | T13.1 20.35,56.95 | 20.35,56.95 v20.7,56.6
+3V3  (via drill 0.2, 0.3)
  Top 0.1: R74.2 v39.58,59.55
  Top 0.2: IC2.9 36.35,56.97 36.52,57.14 v36.73,57.14 | C10.1 32.4,52.7 32.3,52.8 v32.3,54.28 | v77.2,33.59 77.77,33.59 77.94,33.42 L13.1 76.94,32.28 C52.1 | T8.2 73.45,26.95 v73.1,26.6 | R44.2 73.7,35.63 73.87,35.8 v73.87,37.17 74.09,37.39 R70.1 | R71.1 v27.8,59.7 | IC2.1 38.31,53.25 v38.7,52.86
  Top 0.25: IC2.18 33.75,53.25 33.2,52.7 C10.1
  Top 0.305: C15.1 C10.1 | v38.7,52.86 C13.1 39.44,52.5 39.65,52.29 43.42,52.29 44.7,51.01 44.7,48.8 | R75.2 44.29,48.39 44.7,48.8 | v45.4,48.4 45.1,48.4 44.7,48.8
  Top 0.4: R60.2 v20.9,53.6
  Layer2 0.254: v77.4,18.4 75,18.4 73.1,20.3 v73.1,26.6
  Layer2 0.305: v45.4,48.4 45.9,47.9 45.9,46.5 50.3,42.1 52.3,42.1 52.6,41.8 73.1,41.8 v73.2,41.7 73.87,41.03 v73.87,37.17
  Layer2 0.4: v22.64,68.4 26.5,68.4 27.5,67.4 v27.5,66.39 | v33.7,22.1 30.7,22.1 29.51,20.91 v29.51,9.1
  Layer2 0.406: v26.9,50 26.9,51.8 v27.85,52.75 | v32.3,54.28 32.3,55.2 31.3,56.2 30.6,56.2 27.8,59 v27.8,59.7 | v27.5,66.39 33.9,59.99 33.9,58.9 34.9,57.9 36.1,57.9 36.73,57.27 v36.73,57.14
  Layer3 0.1: v16,68.25 16.35,68.25 16.7,68.6 22.44,68.6 v22.64,68.4
  Layer3 0.161: 74.97,33.6 74.91,33.6 74.9,33.59
  Layer3 0.2: v77.2,33.59 74.9,33.59 74.77,33.59 72,30.82 72,27 72.4,26.6 v73.1,26.6 | v73.87,37.17 73.87,34.7 74.97,33.6
  Layer3 0.254: v90.9,16.6 90.1,17.4 81.8,17.4 80.8,18.4 v77.4,18.4
  Layer3 0.4: 30.8,33.4 v33.7,30.5
  Layer3 0.406: 30.8,33.4 v30.8,39.5 30.8,40.6 32.5,42.3 | v33.7,22.1 v33.7,30.5 | v11.6,50.4 14.8,53.6 v20.9,53.6 23.3,53.6 v26.9,50 | v22.64,68.4 23.7,68.4 24.7,67.4 24.7,66.6 27,64.3 27,60.7 27.8,59.9 v27.8,59.7
  Bottom 0.1: C30.1 34.44,29.45 34.16,29.18 IC6.16 | IC5.16 33.98,20.77 34.45,21.25 C27.1 | R30.2 C36.1 | R63.2 v16,68.25
  Bottom 0.2: v36.73,57.14 C3.1 C12.1 C9.1 39.34,57.84 39.58,58.08 v39.58,59.55 | IC7.5 C22.1 | IC9.1 v27.5,66.39 | v22.64,68.4 C46.1 | R30.2 v73.87,37.17 | R26.1 v77.2,33.59 | v29.51,9.1 12.01,9.1 10.76,10.35 8.06,10.35 | 8.06,10.35 D10.2 | D10.1 8.1,8.45 8.35,8.7 8.35,10.06 8.06,10.35
  Bottom 0.254: L18.2 96.3,16.1 96.1,15.9 91.6,15.9 v90.9,16.6
  Bottom 0.305: v73.2,41.7 73.2,40.64 T3.2
  Bottom 0.4: v27.85,52.75 30.11,52.75 v30.64,53.28 | v26.9,50 29.4,50 v30.55,48.85 | v32.3,54.28 32.3,54.2 31.9,53.8 31.3,53.8 | L8.1 v29.51,9.1
  Bottom 0.406: IC7.5 v30.8,39.5 | C30.1 v33.7,30.5 | C27.1 v33.7,22.1 | v30.64,53.28 31.16,53.8 31.3,53.8
  other vias: 11.6,49.6 11.6,48.8 11.6,48 12.4,48.8 13.2,48.8 12.4,48 13.2,48 13.2,47.2 12.4,47.2 13.2,46.4 12.4,46.4 11.6,47.2 11.6,46.4 11.6,51.2 11.6,52 11.6,52.8 11.6,53.6
  pour Top (no thermals): 14.6,55.1 12.2,55.1 11,53.9 11,46.5 11.7,45.8 15,45.8 15.2,46 15.2,49.8 15,50 15,54.7
  pour Layer3: 39.8,60.1 27.8,60.1 25.9,58.2 15.8,58.2 10.7,53.1 10.7,46.5 13,44.2 29.8,44.2 32.2,41.8 40.4,41.8 40.7,42.1 40.7,44.6 41.6,45.5 45.5,45.5 46.3,46.3 46.3,48.7 45.2,49.8 41.7,49.8 40,51.5 40,59.9
+3V3_CPU  (via drill 0.2)
  Top 0.1: R48.2 v65.35,48.8 | v73.55,47.6 R47.1
  Top 0.2: J2.1 5.43,10.76 v5.19,11 | R53.1 v17.47,61.8 | PCORE_.J2-52 43.99,41.91 v44.3,41.6
  Top 0.25: v35.4,35.5 31.8,35.5 30.2,33.9 30.2,29.8 30.9,30.5 v32.52,30.5
  Top 0.254: v9.88,15.21 R11.2 R9.2 | 30.2,29.8 30.2,18.86 v30.25,18.81
  Top 0.305: R7.1 R6.1 v91.3,10.85
  Top 0.4: R4.1 v80.5,11.09
  Layer2 0.1: v73.55,47.6 72.55,48.6 65.55,48.6 v65.35,48.8
  Layer2 0.25: v44.3,41.6 43.2,42.7 39.6,42.7 32.9,49.4 32.8,49.4 32.8,52.3 29.3,55.8 23.6,55.8 22.4,57 22.4,61.9 22,62.3 17.97,62.3 v17.47,61.8 | 12.8,61.8 11.8,60.8 11.8,56.5 13,55.3 17.2,55.3 17.8,54.7 17.8,44.6 18.6,43.8 27.3,43.8 35.4,35.7 v35.4,35.5
  Layer2 0.254: 12.8,61.8 13.1,62.1 17.17,62.1 v17.47,61.8
  Layer2 0.406: v31.2,13.9 31.2,17.86 v30.25,18.81
  Layer3 0.1: v44.3,41.6 46.1,41.6 46.6,42.1 63.7,42.1 65.35,43.75 v65.35,48.8 | v14.6,68.25 14.6,64.67 v17.47,61.8
  Layer3 0.406: v30.25,16.91 v30.25,18.81
  Bottom 0.1: R67.2 v14.6,68.25
  Bottom 0.2: v35.4,35.5 35.45,35.5 | R5.1 v32.52,30.5 | R80.2 19.18,57.82 18.8,58.2 17.7,58.2 17.47,58.43 v17.47,61.8
  Bottom 0.305: v91.3,10.85 90.75,10.3 81.29,10.3 v80.5,11.09
  Bottom 0.4: R2.1 v30.25,18.81 | v80.5,11.09 60.61,11.09 58.6,13.1 32,13.1
  Bottom 0.406: 9.9,11.9 12.2,9.6 28.5,9.6 32,13.1 v31.2,13.9 | 9.9,11.9 9.9,15.19 v9.88,15.21 9.51,14.84 R8.2 | 9.9,11.9 9.4,11.4 5.59,11.4 v5.19,11 | R3.1 v30.25,16.91
+5VS  (via drill 0.2, 0.2 pad 0.25)
  Top 0.2: C17.2 40.48,47.48 39.9,46.9 38,46.9 37.7,46.6 v37.7,46.1 | IC15.1 25.32,49.4 v25.72,49.4
  Top 0.254: J12.18 v89.67,32.08
  Top 0.4: R57.2 27.75,45.48 27.85,45.38 v27.85,44.78 28.3,44.33 v28.3,36.6
  Layer2 0.2: v34.1,56.8 34.1,49 37,46.1 v37.7,46.1 | 61.5,37.2 44.6,37.2 44.3,36.9 44.3,34.1 43.91,33.71 v40.46,33.71 36.99,33.71 36,34.7 v36,37
  Layer2 0.254: v89.67,32.08 83.08,32.08 80.7,29.7 78.1,29.7 75.6,27.2 71.5,27.2 61.5,37.2
  Layer3 0.1: v27.9,55.2 23.3,55.2 21.7,56.8 21.7,61.1 20.6,62.2 17.4,62.2 14.8,64.8 14.8,66.2 16.3,67.7 16.85,67.7 v17.4,68.25
  Layer3 0.2: v37.7,46.1 36.6,47.2 35.7,47.2 34.6,48.3 31.7,48.3 v30.8,47.4 | v27.9,55.2 27.4,54.7 27.4,49.8 27,49.4 v25.72,49.4
  Layer3 0.4: v29.5,7.4 29.1,7.4 28.7,7.8 28.7,36.2 v28.3,36.6
  Bottom 0.1: IC18.5 R79.2 | R65.2 v17.4,68.25
  Bottom 0.2: v27.85,44.78 R62.2 | v37.7,46.1 38,46.1 38.27,45.84 IC4.7 | v25.72,49.4 27.55,49.4 27.85,49.1 C65.1 | F1.1 29.79,47.09 30.1,47.4 v30.8,47.4 | 25.1,54.8 27.5,54.8 v27.9,55.2 | R81.1 34.25,56.65 v34.1,56.8
  Bottom 0.305: R82.2 C76.2 25.1,54.8 24.9,55 IC18.5
  Bottom 0.4: 31.65,34.55 C33.1 28.55,34.55 28.3,34.8 v28.3,36.6 | 31.65,34.55 32.06,34.13 IC7.3 | C65.1 C66.1 R62.2 F1.1 | 31.65,34.55 32.6,35.5 34.3,35.5 35.8,37 v36,37 | L9.2 v29.5,7.4
AUDIO_A_GND  (via drill 0.2)
  Top 0.161: v40.7,46.3 40.39,45.99 PCORE_.J2-69
  Top 0.305: R40.2 32.8,58.2 v32.7,58.3 32.09,58.3 J11.1
  Top 0.4: J11.1 30.69,64.68 v30.71,64.7
  Layer3 0.305: v32.7,58.3 32.9,58.1 32.9,52.1 38,47 40.3,47 40.7,46.6 v40.7,46.3
  Bottom 0.2: v30.71,64.7 D5.3 IC9.2 C51.2 | v30.71,64.7 C50.2 33.81,63.96 34.12,63.65 37,63.65 R42.1 37.5,63.45 37.7,63.65 37.7,65.3 37.2,65.8 R41.2 37.55,66.8 38.63,66.8 C48.2 | 30.3,68.1 D6.3 | v30.72,64.71 v30.71,64.7 | D6.1 33.5,69.1 33.82,68.78 C49.1
  Bottom 0.305: v30.72,64.71 30.72,67.68 30.3,68.1 30.7,68.5 30.7,68.98 30.82,69.1 D6.1
AUDIO_A_HP_L  (via drill 0.2)
  Top 0.2: v35.3,46 35.3,42.1 36.2,41.2 38.9,41.2 39.19,41.49 PCORE_.J2-76
  Layer3 0.2: v35.3,46 31.6,46 30.1,47.5 30.1,58.6 32.7,61.2 36.2,61.2 36.6,61.6 36.6,64.5 36,65.1 v36,67.29 v35.99,67.3
  Bottom 0.2: v35.99,67.3 C44.1
AUDIO_A_HP_R  (via drill 0.2)
  Top 0.2: PCORE_.J2-78 38.79,41.79 38.6,41.6 36.3,41.6 35.7,42.2 v35.7,45.5
  Layer3 0.2: v36.06,61.8 35.96,61.7 32.6,61.7 29.7,58.8 29.7,47.3 31.4,45.6 35.2,45.6 35.3,45.5 v35.7,45.5
  Bottom 0.2: v36.06,61.8 C45.1
AUDIO_A_IN_L  (via drill 0.2)
  Top 0.2: v38.79,46.15 PCORE_.J2-77 | J9.48 32.23,1.73 33.5,3 33.5,5.6 32.8,6.3 32.8,10.7 v33.7,11.6
  Layer3 0.2: v38.79,46.15 38.79,35.71 39.8,34.7 41.2,34.7 42.5,33.4 42.5,15.8 40.6,13.9 35,13.9 33.7,12.6 v33.7,11.6
AUDIO_A_IN_R  (via drill 0.2)
  Top 0.2: J9.44 36,3 36,5.2 35.4,5.8 34.6,5.8 33.7,6.7 v33.7,10.4
  Top 0.23: v38.32,46.45 38.32,45.78 38.39,45.71 PCORE_.J2-79
  Layer3 0.2: v38.32,46.45 38.32,35.68 39.7,34.3 41,34.3 42.1,33.2 42.1,16 40.4,14.3 34.8,14.3 33.3,12.8 33.3,10.8 v33.7,10.4
AUDIO_A_MIC  (via drill 0.2)
  Top 0.2: v36.2,44.9 36.8,44.3 39,44.3 39.19,44.49 PCORE_.J2-75 v39.19,46.45 | J9.41 39.8,5.3 38.9,6.2 34.8,6.2 34.2,6.8 v34.2,10.7
  Layer3 0.2: v39.7,66.2 38.1,67.8 35.9,67.8 32.2,64.1 32.2,61.9 29.3,59 29.3,47.2 31.3,45.2 35.2,45.2 35.5,44.9 v36.2,44.9 | v34.2,10.7 34.2,12.4 35.3,13.5 40.8,13.5 42.9,15.6 42.9,33.6 41.4,35.1 40,35.1 39.19,35.91 v39.19,46.45
  Bottom 0.2: L12.1 C48.1 v39.7,66.2
AUDIO_A_OUT_L  (via drill 0.2)
  Top 0.2: v39.99,46.45 PCORE_.J2-71 | J9.49 29.64,4.34 31,5.7 31.9,5.7 32.4,6.2 32.4,11 33.5,12.1 v35.3,12.1
  Layer3 0.2: v39.99,46.45 39.99,36.31 40.4,35.9 41.8,35.9 43.7,34 43.7,15.3 41.1,12.7 35.9,12.7 v35.3,12.1
AUDIO_A_OUT_R  (via drill 0.2)
  Top 0.2: v39.59,46.13 PCORE_.J2-73 | J9.45 34.72,5.08 33.2,6.6 33.2,10.5 33.9,11.2 v34.7,11.2
  Layer3 0.2: v39.59,46.13 39.59,36.11 40.2,35.5 41.6,35.5 43.3,33.8 43.3,15.4 41,13.1 35.6,13.1 34.7,12.2 v34.7,11.2
AUDIO_A_VCC  (via drill 0.2)
  Top 0.2: PCORE_.J2-67 40.79,44.69 40,43.9 36.5,43.9 v36.2,44.2
  Layer3 0.2: v23.68,66.49 22.6,65.41 22.6,61.7 22,61.1 22,58.4 22.7,57.7 28.3,57.7 28.9,57.1 28.9,47.1 31.2,44.8 35,44.8 35.6,44.2 v36.2,44.2
  Bottom 0.2: IC9.5 C51.1 v23.68,66.49
B0  (via drill 0.2)
  Top 0.1: v86.4,33.35 J12.16
  Bottom 0.1: IC12.4 88.35,29.45 86.6,31.2 86.6,33.15 v86.4,33.35
B1  (via drill 0.2)
  Top 0.1: v85.6,33.35 J12.15
  Bottom 0.1: IC10.11 84.15,28.05 85.2,29.1 85.2,32.95 v85.6,33.35
B2  (via drill 0.2)
  Top 0.1: v86.4,19.38 J12.38
  Bottom 0.1: IC13.3 88.41,21.12 86.67,19.38 v86.4,19.38
B3  (via drill 0.2)
  Top 0.1: v85.6,18.11 J12.39
  Bottom 0.1: IC11.13 83.34,15.85 v85.6,18.11
B4  (via drill 0.2)
  Top 0.1: v86.4,18.11 J12.40
  Bottom 0.1: IC13.2 88.47,20.72 86.93,19.18 86.93,18.64 v86.4,18.11
B5  (via drill 0.2)
  Top 0.1: v85.6,16.84 J12.41
  Bottom 0.1: IC11.14 84.21,15.45 v85.6,16.84
B6  (via drill 0.2)
  Top 0.1: v86.4,16.84 J12.42
  Bottom 0.1: IC13.1 88.52,20.32 87.2,19 87.2,17.64 v86.4,16.84
B7  (via drill 0.2)
  Top 0.1: v85.6,15.57 J12.43
  Bottom 0.1: IC11.15 85.08,15.05 v85.6,15.57
BL_PWM  (via drill 0.2)
  Top 0.1: PCORE_.J1-48 v48.59,7.45 | v82.4,42.24 J12.1
  Layer3 0.1: v48.59,7.45 48.59,8.49 48.8,8.7 49.9,8.7 51.4,10.2 51.4,12.2 52.2,13 74.7,13 75.2,12.5 78.5,12.5 79,12 84.4,12 85.1,11.3 88.3,11.3 93.8,16.8 93.8,34.3 87.7,40.4 84.24,40.4 v82.4,42.24
BTN_ON/OFF  (via drill 0.2, 0.2 pad 0.25)
  Top 0.1: v49.39,7.45 PCORE_.J1-44 | T10.21 2.4,28.1 2.8,28.1 2.9,28 v4.4,28 5.7,26.7 v7.4,26.7
  Layer2 0.1: v3.4,16.6 2.7,16.6 2.3,17 2.3,25.9 v4.4,28
  Layer3 0.1: v3.4,16.6 3.4,10.2 5,8.6 9.1,8.6 12.5,5.2 47.8,5.2 49.39,6.79 v49.39,7.45 | v10.8,65.3 10.5,65.3 9.9,64.7 9.9,58.2 8.9,57.2 6.8,57.2 5.4,55.8 5.4,44.8 8.9,41.3 8.9,35.1 6.7,32.9 6.7,27.4 v7.4,26.7
  Bottom 0.1: R17.2 v10.8,65.3
CAN1H
  Bottom 0.2: IC7.7 33.34,39.37 33.2,39.5 R20.1 33.2,40.6 32.6,41.2 29.7,41.2 28.7,40.2 25.68,40.2 25.2,40.67 25.2,41.7 24.5,42.4 23.6,42.4 22.9,41.7 22.9,40.7 24.04,39.56 J5.4
CAN1L
  Bottom 0.2: IC7.6 32.06,39.37 32.2,39.5 R20.2 32.2,40.6 32,40.8 29.9,40.8 28.9,39.8 25.51,39.8 J5.3
CAN_A_RX  (via drill 0.2)
  Top 0.1: PCORE_.J1-10 v56.19,7.45
  Layer2 0.1: v56.19,7.45 56.19,6.79 55.4,6 41.5,6 41.1,6.4 41.1,12.2 35.2,18.1 35.2,22.4 30.8,26.8 v30.8,31.3
  Bottom 0.1: IC7.4 v30.8,31.3 R5.2
CAN_A_TX  (via drill 0.2)
  Top 0.1: PCORE_.J1-12 v55.79,7.15
  Layer2 0.1: v55.79,7.15 55.79,6.79 55.2,6.2 41.6,6.2 41.3,6.5 41.3,12.3 35.4,18.2 35.4,22.5 31,26.9 31,30.7 31.6,31.3 v34.6,31.3
  Bottom 0.1: v34.6,31.3 IC7.1
CLK  (via drill 0.2)
  Top 0.1: v86.4,30.8 J12.20
  Bottom 0.1: IC12.3 88.25,29.05 86.5,30.8 v86.4,30.8
CTS_C_RS232
  Bottom 0.1: IC6.8 35.83,24.62 34.8,23.6 31.5,23.6 30.6,24.5 30.6,26.8 30.1,27.3 26.1,27.3 24.8,28.6 22.63,28.6 J8.6
DE  (via drill 0.2)
  Top 0.1: J12.45 85.3,14.3 v85.6,14.6
  Bottom 0.1: IC11.16 85.55,14.65 v85.6,14.6
ETH_A_D1_N  (via drill 0.2)
  Top 0.127: PCORE_.J2-3 53.69,45.34 53.69,46.15 53.95,46.41 54.75,46.41 55.01,46.15 55.01,45.3 v55.15,45.3
  Bottom 0.127: v55.15,45.3 55.01,45.3 55.01,44.45 54.75,44.19 52.55,44.19 52.41,44.05 52.41,43.85 52.55,43.71 54.85,43.71 55.11,43.45 55.11,43.05 54.85,42.79 52.65,42.79 52.51,42.65 52.51,42.45 52.65,42.31 55.45,42.31 55.59,42.45 55.59,46.25 57.45,48.11 66.9,48.11 67.64,48.85 67.64,50.25 69.7,52.31 76.7,52.31 77.54,53.15 77.54,56.92 J15.L1
ETH_A_D1_P  (via drill 0.2)
  Top 0.127: PCORE_.J2-1 53.91,45.32 53.91,46.05 54.05,46.19 54.65,46.19 54.79,46.05 54.79,45.3 v54.65,45.3
  Bottom 0.127: v54.65,45.3 54.79,45.3 54.79,44.55 54.65,44.41 52.45,44.41 52.19,44.15 52.19,43.75 52.45,43.49 54.75,43.49 54.89,43.35 54.89,43.15 54.75,43.01 52.55,43.01 52.29,42.75 52.29,42.35 52.55,42.09 55.55,42.09 55.81,42.35 55.81,46.15 57.55,47.89 67,47.89 67.86,48.75 67.86,50.15 69.8,52.09 76.8,52.09 77.76,53.05 77.76,55.1 77.96,55.3 78.55,55.3 78.79,55.06 J15.L2
ETH_A_D2_N  (via drill 0.2)
  Top 0.127: PCORE_.J2-7 52.89,45.34 52.89,46.45 53.65,47.21 57.15,47.21 57.71,46.65 57.71,45.3 v57.85,45.3
  Bottom 0.127: v57.85,45.3 57.71,45.3 57.71,43.85 57.45,43.59 56.85,43.59 56.71,43.45 56.71,43.35 56.85,43.21 57.75,43.21 58.01,42.95 58.01,42.65 57.75,42.39 56.85,42.39 56.71,42.25 56.71,42.15 56.85,42.01 58.05,42.01 58.39,42.35 58.39,46.25 59.15,47.01 67.9,47.01 68.84,47.95 68.84,49.75 70.6,51.51 78.9,51.51 80.04,52.65 80.04,56.92 J15.L3
ETH_A_D2_P  (via drill 0.2)
  Top 0.127: PCORE_.J2-5 53.11,45.32 53.11,46.35 53.75,46.99 57.05,46.99 57.49,46.55 57.49,45.3 v57.35,45.3
  Bottom 0.127: v57.35,45.3 57.49,45.3 57.49,43.95 57.35,43.81 56.75,43.81 56.49,43.55 56.49,43.25 56.75,42.99 57.65,42.99 57.79,42.85 57.79,42.75 57.65,42.61 56.75,42.61 56.49,42.35 56.49,42.05 56.75,41.79 58.15,41.79 58.61,42.25 58.61,46.15 59.25,46.79 68,46.79 69.06,47.85 69.06,49.65 70.7,51.29 79,51.29 80.26,52.55 80.26,55.2 80.46,55.4 81.15,55.4 81.33,55.22 J15.L4
ETH_A_D3_N  (via drill 0.2)
  Top 0.127: PCORE_.J2-11 52.09,45.34 52.09,46.85 53.15,47.91 59.45,47.91 60.31,47.05 60.31,45.3 v60.45,45.3
  Bottom 0.127: v60.45,45.3 60.31,45.3 60.31,44.85 60.05,44.59 59.85,44.59 59.71,44.45 59.71,44.35 59.85,44.21 60.15,44.21 60.41,43.95 60.41,43.65 60.15,43.39 59.85,43.39 59.71,43.25 59.71,43.15 59.85,43.01 60.65,43.01 60.89,43.25 60.89,45.25 61.55,45.91 68.9,45.91 70.34,47.35 70.34,49.55 71.5,50.71 80.5,50.71 82.54,52.75 82.54,56.88 J15.L5
ETH_A_D3_P  (via drill 0.2)
  Top 0.127: PCORE_.J2-9 52.31,45.32 52.31,46.75 53.25,47.69 59.35,47.69 60.09,46.95 60.09,45.3 v59.95,45.3
  Bottom 0.127: v59.95,45.3 60.09,45.3 60.09,44.95 59.95,44.81 59.75,44.81 59.49,44.55 59.49,44.25 59.75,43.99 60.05,43.99 60.19,43.85 60.19,43.75 60.05,43.61 59.75,43.61 59.49,43.35 59.49,43.05 59.75,42.79 60.75,42.79 61.11,43.15 61.11,45.15 61.65,45.69 69,45.69 70.56,47.25 70.56,49.45 71.6,50.49 80.6,50.49 82.76,52.65 82.76,55.2 82.96,55.4 83.65,55.4 83.87,55.18 J15.L6
ETH_A_D4_N
  Top 0.127: PCORE_.J2-15 51.29,45.34 51.29,47.25 55.15,51.11 73.5,51.11 73.64,51.25 73.64,52.95 73.9,53.21 74.3,53.21 74.56,52.95 74.56,51.25 74.7,51.11 74.9,51.11 75.04,51.25 75.04,52.95 75.3,53.21 75.7,53.21 75.96,52.95 75.96,51.35 76.1,51.21 83.8,51.21 85.14,52.55 J15.L7
ETH_A_D4_P
  Top 0.127: PCORE_.J2-13 51.51,45.32 51.51,47.15 55.25,50.89 73.6,50.89 73.86,51.15 73.86,52.85 74,52.99 74.2,52.99 74.34,52.85 74.34,51.15 74.6,50.89 75,50.89 75.26,51.15 75.26,52.85 75.4,52.99 75.6,52.99 75.74,52.85 75.74,51.25 76,50.99 83.9,50.99 85.36,52.45 85.36,55.2 85.56,55.4 86.15,55.4 86.41,55.14 J15.L8
ETH_B_D1_N
  Top 0.127: PCORE_.J2-21 50.09,45.34 50.09,47.35 55.05,52.31 59.3,52.31 59.44,52.45 59.44,54.15 59.7,54.41 60.1,54.41 60.36,54.15 60.36,52.45 60.5,52.31 60.7,52.31 60.84,52.45 60.84,54.45 61.1,54.71 61.5,54.71 61.76,54.45 61.76,52.45 61.9,52.31 62.1,52.31 62.24,52.45 62.24,54.45 62.5,54.71 62.9,54.71 63.16,54.45 63.16,52.45 63.3,52.31 63.4,52.31 63.54,52.45 63.54,56.93 J15.R1
ETH_B_D1_P
  Top 0.127: PCORE_.J2-19 50.31,45.32 50.31,47.25 55.15,52.09 59.4,52.09 59.66,52.35 59.66,54.05 59.8,54.19 60,54.19 60.14,54.05 60.14,52.35 60.4,52.09 60.8,52.09 61.06,52.35 61.06,54.35 61.2,54.49 61.4,54.49 61.54,54.35 61.54,52.35 61.8,52.09 62.2,52.09 62.46,52.35 62.46,54.35 62.6,54.49 62.8,54.49 62.94,54.35 62.94,52.35 63.2,52.09 63.5,52.09 63.76,52.35 63.76,55.08 63.95,55.27 64.62,55.27 64.82,55.07 J15.R2
ETH_B_D2_N  (via drill 0.2)
  Top 0.127: v47.3,49.95 47.3,50.09 47.95,50.09 49.29,48.75 49.29,45.34 PCORE_.J2-25
  Bottom 0.127: v47.3,49.95 47.3,50.09 46.85,50.09 46.59,50.35 46.59,50.85 46.85,51.11 48.45,51.11 48.71,50.85 48.71,50.25 48.85,50.11 48.95,50.11 49.09,50.25 49.09,50.95 49.35,51.21 49.65,51.21 49.91,50.95 49.91,50.25 50.05,50.11 53.25,50.11 56.45,53.31 65.6,53.31 66.18,53.89 66.18,56.85 J15.R3
ETH_B_D2_P  (via drill 0.2)
  Top 0.127: v47.3,50.45 47.3,50.31 48.05,50.31 49.51,48.85 49.51,45.32 PCORE_.J2-23
  Bottom 0.127: v47.3,50.45 47.3,50.31 46.95,50.31 46.81,50.45 46.81,50.75 46.95,50.89 48.35,50.89 48.49,50.75 48.49,50.15 48.75,49.89 49.05,49.89 49.31,50.15 49.31,50.85 49.45,50.99 49.55,50.99 49.69,50.85 49.69,50.15 49.95,49.89 53.35,49.89 56.55,53.09 65.7,53.09 66.4,53.79 66.4,55.25 66.55,55.4 67.25,55.4 67.36,55.29 J15.R4
ETH_B_D3_N  (via drill 0.2)
  Top 0.127: PCORE_.J2-29 48.49,45.34 48.49,47.45 47.65,48.29 47.3,48.29 v47.3,48.15
  Bottom 0.127: v47.3,48.15 47.3,48.29 46.85,48.29 46.59,48.55 46.59,48.95 46.85,49.21 48.25,49.21 48.51,48.95 48.51,48.35 48.65,48.21 48.75,48.21 48.89,48.35 48.89,48.85 49.15,49.11 49.45,49.11 49.71,48.85 49.71,48.35 49.85,48.21 53.05,48.21 57.05,52.21 66.6,52.21 68.64,54.25 J15.R5
ETH_B_D3_P  (via drill 0.2)
  Top 0.127: PCORE_.J2-27 48.71,45.32 48.71,47.55 47.75,48.51 47.3,48.51 v47.3,48.65
  Bottom 0.127: v47.3,48.65 47.3,48.51 46.95,48.51 46.81,48.65 46.81,48.85 46.95,48.99 48.15,48.99 48.29,48.85 48.29,48.25 48.55,47.99 48.85,47.99 49.11,48.25 49.11,48.75 49.25,48.89 49.35,48.89 49.49,48.75 49.49,48.25 49.75,47.99 53.15,47.99 57.15,51.99 66.7,51.99 68.86,54.15 68.86,55.11 69.05,55.3 69.75,55.3 69.9,55.15 J15.R6
ETH_B_D4_N  (via drill 0.2)
  Top 0.127: PCORE_.J2-33 47.69,45.34 47.69,46.35 47.55,46.49 47.3,46.49 v47.3,46.35
  Bottom 0.127: v47.3,46.35 47.3,46.49 47.05,46.49 46.91,46.35 46.91,46.15 47.05,46.01 52.55,46.01 57.55,51.01 67,51.01 69.2,53.21 70.4,53.21 71.14,53.95 71.14,56.91 J15.R7
ETH_B_D4_P  (via drill 0.2)
  Top 0.127: PCORE_.J2-31 47.91,45.32 47.91,46.45 47.65,46.71 47.3,46.71 v47.3,46.85
  Bottom 0.127: v47.3,46.85 47.3,46.71 46.95,46.71 46.69,46.45 46.69,46.05 46.95,45.79 52.65,45.79 57.65,50.79 67.1,50.79 69.3,52.99 70.5,52.99 71.36,53.85 71.36,55.11 71.55,55.3 72.25,55.3 72.44,55.11 J15.R8
G0  (via drill 0.2)
  Top 0.1: v85.6,34.62 J12.13
  Bottom 0.1: IC10.10 84.15,28.45 84.9,29.2 84.9,33.92 v85.6,34.62
G1  (via drill 0.2)
  Top 0.1: v86.4,34.62 J12.14
  Bottom 0.1: IC12.5 88.45,29.85 87,31.3 87,34.02 v86.4,34.62
G2  (via drill 0.2)
  Top 0.1: v85.6,23.19 J12.31
  Bottom 0.1: IC11.10 82.95,17.05 84.3,18.4 84.3,21.89 v85.6,23.19
G3  (via drill 0.2)
  Top 0.1: v86.4,23.19 J12.32
  Bottom 0.1: IC13.6 87.96,22.32 87.09,23.19 v86.4,23.19
G4  (via drill 0.2)
  Top 0.1: v85.6,21.92 J12.33
  Bottom 0.1: IC11.11 83.05,16.65 84.7,18.3 84.7,21.02 v85.6,21.92
G5  (via drill 0.2)
  Top 0.1: v86.4,21.92 J12.34
  Bottom 0.1: IC13.5 v86.4,21.92
G6  (via drill 0.2)
  Top 0.1: v85.6,20.65 J12.35
  Bottom 0.1: IC11.12 83.15,16.25 85,18.1 85,20.05 v85.6,20.65
G7  (via drill 0.2)
  Top 0.1: v86.4,20.65 J12.36
  Bottom 0.1: IC13.4 88.28,21.52 87.41,20.65 v86.4,20.65
GND  (via drill 0.2, 0.2 pad 0.25, 0.3)
  Top 0.127: C54.2 95.01,55.93 R1.2 | C55.2 v59.78,55.26
  Top 0.15: v21.35,60.1 C64.2 20.4,60.3 20.1,60.6 18.6,60.6 18.43,60.77 C63.2
  Top 0.2: IC15.9 24.8,47.4 v24.9,47.5 | C13.2 41.31,52.86 v41.46,53.01 | v42.79,46.23 PCORE_.J2-57 42.79,44.61 43,44.4 44.5,44.4 44.79,44.69 PCORE_.J2-47 | PCORE_.J1-62 v45.79,7.15 | PCORE_.J1-63 v45.39,11.84 | v48.99,7.15 PCORE_.J1-46 PCORE_.J1-45 | PCORE_.J2-74 39.59,43.34 39.44,43.5 37.59,43.5 37.33,43.24 v37.33,42.5 | R34.1 C39.2 96.58,28.5 v96.63,28.45 | v74.9,34.43 74.9,33.5 75.04,33.36 T7.2 | C53.2 80.71,37.95 80.9,37.76 v81.25,37.76 | R46.1 v76.3,36.1 | PCORE_.J1-52 v47.79,7.45 | v39.79,51.05 39.59,51.25 C5.1 39,50.2 BQ1.2 | PCORE_.J2-17 v50.79,44.22 | C56.2 v3.6,29.85 | PCORE_.J2-35 47.19,44.3 v47.6,43.89 | C6.1 36.4,49 36.6,48.8 36.8,48.8 37.2,48.4 BQ1.4 | J1.5 v21.9,66.1
  Top 0.23: PCORE_.J1-80 42.19,7.52 v42.12,7.45
  Top 0.25: IC15.3 v24.3,48.5 | v4.4,16.4 4.4,17.29 R56.1
  Top 0.254: IC2.6 37.35,55.75 v36.8,55.2 | v42.12,7.46 v42.12,7.45 | J16.6 v94.84,13.47 v94.85,13.47
  Top 0.305: C60.2 21.25,48.6 C59.2 19.85,47.9 19.6,48.15 19.6,50.6 20.25,51.25 R54.1 R61.1 | C15.2 C10.2 R14.1 31.8,54.3 v31.7,54.4 | R40.1 R13.1
  Top 0.4: J12.19 v85.6,30.81 | J12.23 v85.6,28.27 | J12.37 v85.6,19.38 | v86.4,24.46 J12.30 | C14.2 R15.1 v42.2,50.25 | C60.2 v22.5,48.6 | R58.1 v23.8,43.15 | T9.2 v14.2,60.85 | C68.2 v17.2,47.1 | C67.2 v16.5,48.5 | v31.11,55.25 R12.1 R13.1 | v42.56,47.48 C17.1 | J2.3 v5.29,12.03 | J2.9 7.5,15.84 v8.19,16.53 | C37.2 v93.63,40.65 | C6.1 v35.95,48.35 | v5.29,13.3 J2.5 | T11.11 v10.5,1.6 | T12.11 v21.3,1.6
  Top 0.406: J12.9 v82.35,37.16 | J12.44 v86.45,15.57 | C61.2 v14.54,56.22 | C62.2 v15.66,57.18 | LED3.C v14,71.5 | LED1.C v15.4,71.5 | LED2.C v16.8,71.5
  Bottom 0.1: R18.1 v8.6,65.4 | v21.35,60.1 21.35,58.5 21.65,58.2 T13.2 21.65,56.95 21.9,56.7 23.2,56.7 23.4,56.9 23.4,57.4 23.9,57.9 D11.2
  Bottom 0.2: T2.2 C38.2 v78.05,34.7 | v21.8,61.75 21.8,64.5 22,64.7 C47.2 C46.2 22.15,65.85 v21.9,66.1 | C43.2 C42.2 v80,41.06 | v77,37.76 T4.2 | R35.1 C40.2 C41.2 v75.05,23.77 | IC8.2 v74.9,34.43 | v71.65,33.55 C34.2 C35.2 | v72.75,32.15 R33.1 | T6.2 v96.63,28.45 | IC17.2 45.7,34.48 v45.99,34.19 | v48.67,35.96 C73.2 48.01,37.05 48,37.06 C74.2 | D4.3 v77.69,41.77 | v27.9,54.3 26.62,54.3 C76.1 | C78.1 C79.1 v26.38,60.3 | v31.1,57.2 31.25,57.35 T15.2 32.05,56.75 32.2,56.6 R78.1 C80.1 | C75.- v19.2,61.7 | C21.1 41.42,53.05 v41.46,53.01
  Bottom 0.25: 4,16 C69.2 4,16.3 4.1,16.4 v4.4,16.4 | v19.8,55.4 19.3,55.4 19.18,55.28 C77.1 18.7,54.95 18.5,55.15 v18.5,56.8
  Bottom 0.254: C71.2 v95.07,16.77
  Bottom 0.305: v34.75,59.53 C11.2 | C8.2 v35.74,59.53 | C3.2 v36.73,59.53 | C12.2 v37.73,59.53 | C9.2 v38.74,59.53 | J4.4 J4.8 v46,56.23 | J10.10@1 85.34,38.35 v85.95,38.96 | J10.10@2 v84.5,45.35 | v17.2,47.1 17.8,47.7 C57.2 20.05,47.7 20.95,48.6 v22.5,48.6 | IC18.2 23.9,52.2 24.1,52 25.8,52 26.12,52.32 C76.1 | v45.39,37.99 45.7,38.3 C72.2 | IC16.3 7.2,18.05 C70.2
  Bottom 0.4: C18.- v33.2,47.31 | C65.2 v26.09,48.6 26.09,47.56 C66.2 | C20.1 36.5,53.5 v36.8,53.8 | J10.6 v96.16,42.75 | v95.11,31.48 R25.2 | C22.2 v29.3,36.29 | C33.2 v29.3,36.29 | IC7.2 v33.34,34.3 v33.33,34.3 | C30.2 v36.15,30.5 C31.2 | IC7.8 34.6,36.79 34.1,36.29 v29.3,36.29 | v34.34,28.53 IC6.15 | IC10.17 v80,25.47 | IC12.17 v89.7,27.67 | IC13.17 v89.7,19.78 | v36.7,21.42 C28.2 C27.2 | IC5.15 v34.38,20.12 v34.39,20.12 | C29.2 40.37,15.8 v40.09,15.52 | C32.2 v40.9,23.52 | IC16.3 7.2,16.7 7.4,16.5 8.16,16.5 v8.19,16.53 | IC4.6 39.53,43.03 39,42.5 v37.33,42.5 | IC11.17 v80,17.97
  Bottom 0.406: C19.- v44.6,47.39
  other vias: 12.7,29.8 11.9,29.8 11.1,29.8 10.3,29.8 10.3,30.5 12.7,30.5 11.9,30.5 11.1,30.5 17.8,57.3 17.1,57.3 18.5,57.3 18.5,57.8 17.8,57.8 17.1,57.8 17.1,56.8 17.8,56.8 36.1,54.5 36.8,54.5 36.1,55.2 35.4,55.2 35.4,54.5 35.4,53.8 36.1,53.8 24.3,48 23.7,48 24.9,48 24.9,48.5 23.7,48.5 23.7,47.5 24.3,47.5 51.87,41.62 9.6,29.8 8.8,29.8 8,29.8 8,31.2 8.8,31.2 9.6,30.5 8.8,30.5 8,30.5 9.6,31.2 10.3,31.2 12.7,31.2 11.9,31.2 11.1,31.2 51.28,41.6 52.09,41.16 51.57,41.15 94.91,55.1 95.61,55.1 95.61,54.5 95.61,53.9 94.91,53.9 94.91,54.5 96.31,53.9 97.01,53.9 97.71,53.9
  pour Layer3: 0,43.4 0,0 100,0 100,56.9 99.2,57.7 58.6,57.7 58.4,57.5 58.4,56.7 57.3,55.6 54.8,55.6 53.3,57.1 45.6,57.1 44.2,55.7 40.3,55.7 40.3,51.6 41.9,50.1 45.3,50.1 46.7,48.7 46.7,42.2 46,41.5 32,41.5 29.6,43.9 0.5,43.9
  pour Layer2: 21.7,59.3 21.3,59.3 20.4,60.2 13.2,60.2 12.7,59.7 12.7,58.6 13.1,58.2 18.9,58.2 19,58.1 19,56 17.7,54.5 17.7,47 17.3,46.5 15.5,46.5 15.1,46.1 0.5,46.1 0,46.7 0,61.8 1.3,63.1 20.7,63.1 22,61.8 22,59.6
  pour Top (no thermals): 52.87,40.97 52.87,42.92 52.79,43 52,43 51.91,42.91 51.91,42.27 51.54,41.9 51.2,41.9 51,41.7 51,41.1 51.2,40.9 51.9,40.9
  pour Layer2: 0,72 0,64.6 1.3,63.3 20.9,63.3 22.3,61.9 22.3,59.5 21.8,59 21.2,59 20.3,59.9 13.3,59.9 13,59.6 13,58.7 13.3,58.4 19.1,58.4 19.3,58.2 19.3,56.3 19.5,56.1 21,56.1 21.4,55.7 21.4,47.3 21.9,46.8 28.9,46.8 35.8,39.9 43.9,39.9 44.4,39.3 49.2,39.3 49.6,39.7 51.8,39.7 52.6,38.9 52.6,38 51.9,37.3 33.3,37.3 27,43.6 18.9,43.6 17.6,44.9 17.6,46 17.3,46.3 15.6,46.3 15.2,45.9 0.7,45.9 0,45.2 0,0 100,0 100,72
  pour Top (no thermals): 94.6,56.7 95.9,56.7 96.6,56 97.9,56 98.1,55.8 98.1,53.8 97.9,53.6 94.6,53.6 94.4,53.8 94.4,56.5
  pour Bottom (no thermals): 7.9,29.5 12.8,29.5 13,29.7 13,33.8 12.7,34.1 8,34.1 7.7,33.8 7.7,29.7
  pour Top (no thermals): 7.4,36 7.2,35.8 7.2,30.1 7.8,29.5 12.8,29.5 13,29.7 13,33.8 12.7,34.1 10.4,34.1 10.2,34.3 10.2,35.8 10,36
GND_SHIELD
  pour Bottom (no thermals): 41,72 41,57.2 42.1,56.1 44,56.1 45,57.1 45,62 45.6,62.6 53.6,62.6 54.2,62 54.2,57 55.2,56 56.9,56 57.9,57 57.9,58 58.3,58.4 62.35,58.4 63.25,59.3 63.25,68.1 63.65,68.5 88.65,68.5 89.05,68.1 89.05,59.1 89.65,58.5 93.4,58.5 94,59.1 94,72
  pour Top (no thermals): 17.7,72 17.7,62.5 18,62.2 20.3,62.2 20.6,62.5 20.6,66.2 20.9,66.5 25.8,66.5 26.2,66.1 26.2,62.6 26.5,62.3 30.2,62.3 30.5,62.6 30.5,68.9 31.4,69.8 40.2,69.8 41,69 41,57.2 42.1,56.1 44,56.1 45,57.1 45,62 45.6,62.6 53.6,62.6 54.2,62 54.2,57 55.2,56 56.9,56 57.9,57 57.9,58 58.3,58.4 62.35,58.4 63.25,59.3 63.25,68.1 63.65,68.5 88.65,68.5 89.05,68.1 89.05,59.1 89.65,58.5 93.4,58.5 94,59.1 94,72
  pour Top (no thermals): 93.8,61.3 98,61.3 98.2,61.1 98.2,57.3 98,57.1 96.2,57.1 96,57.3 93.6,57.3 93.4,57.5 93.4,59.1 93.8,59.5
GNDIN  (via drill 0.3)
  other vias: 10.4,41.2 10.4,41.8 10.4,42.4 10.4,43 11,41.8 11,42.4 11,43 11,43.6 10.4,43.6 10.4,44.2 10.4,44.8 11,44.8 11,44.2 9.2,44.8 9.8,44.8 8,44.8 8.6,44.8 7.4,44.8
  pour Top (no thermals): 7.4,45.6 7,45.2 7,40.7 7.2,40.5 10.9,40.5 11.5,41.1 11.5,45.2 11.1,45.6
  pour Bottom (no thermals): 11.5,41.3 10.9,40.7 4.6,40.7 4.1,41.2 4.1,51.3 5.8,53 8.9,53 9.5,52.4 9.5,50.7 8.9,50.1 6.7,50.1 6.3,49.7 6.3,46.1 6.9,45.5 10.9,45.5 11.5,44.9
GPIO_J1_22  (via drill 0.2)
  Top 0.1: PCORE_.J1-22 v53.79,7.45
  Layer3 0.1: v53.79,7.45 53.79,7.79 56.7,10.7 61.7,10.7 64.1,8.3 70.8,8.3 73.9,5.2 84.59,5.2 J9.5
GPIO_J1_24
  Top 0.1: PCORE_.J1-24 53.39,7.21 53.8,6.8 85.53,6.8 J9.3
GPIO_J1_25  (via drill 0.2)
  Top 0.1: PCORE_.J1-25 v52.99,11.85
  Layer3 0.1: v52.99,11.85 52.99,12.51 52.7,12.8 52.3,12.8 51.6,12.1 51.6,6.8 52.7,5.7 57.8,5.7 58.8,4.7 58.8,3.05 J9.26
GPIO_J1_26
  Top 0.1: PCORE_.J1-26 52.99,7.11 53.5,6.6 85,6.6 86.8,4.8 86.8,2.99 J9.4
GPIO_J1_27  (via drill 0.2)
  Top 0.1: PCORE_.J1-27 v52.59,12.25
